FUNCTION "fb_515C_SendData" : VOID
TITLE =Collect the MPI Send signals especial TIE BREAKER
//version!date    !author !change_segm!change_description
//-------+--------+-------+-----------+-------------------------------
// 1.0   !31.08.00!Kahle  ! ---       ! 1st vaild version
// 1.1   !14.11.00!Kahle  ! 1         ! Corr. tie breaker
AUTHOR : Kahle
FAMILY : PMA71
NAME : CollData
VERSION : 1.1


VAR_INPUT
  ONE_TIEBRK : BOOL ;
  IN_Mde_autoOP : BOOL ;	//mode =automatic from OP
END_VAR
VAR_OUTPUT
  IN_Mde_auto : BOOL ;	//mode =automatic from IMAC
END_VAR
VAR_TEMP
  local : BOOL ;	//mode =local
  semiOP : BOOL ;	//mode =semi OP
  autoOP : BOOL ;	//mode =auto OP
  semi : BOOL ;	//mode =semi
  auto : BOOL ;	//mode =auto
  var5 : BOOL ;
  var6 : BOOL ;
  var7 : BOOL ;
END_VAR
BEGIN
NETWORK
TITLE =Collect the MPI Send signals
// c_genBrkOpn, c_unitLock                            ->FB56 "GenProtect"
//
//
// Automatic mode
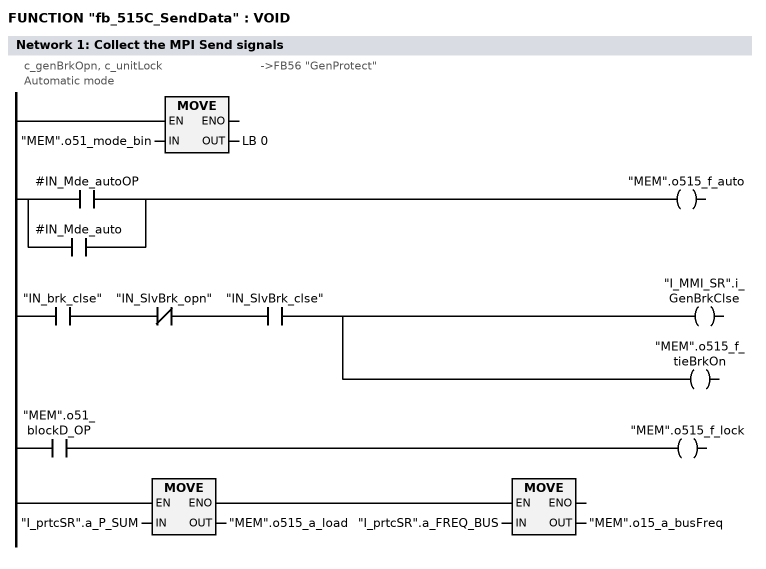
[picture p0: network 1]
      L     "MEM".o51_mode_bin;
      T     LB     0;
      O     #IN_Mde_autoOP;
      O     #IN_Mde_auto;
      =     "MEM".o515_f_auto;

// tie breaker_A close
      U     "IN_brk_clse";
      UN    "IN_SlvBrk_opn";
      U     "IN_SlvBrk_clse";
      =     "I_MMI_SR".i_GenBrkClse;
      =     "MEM".o515_f_tieBrkOn;

// tie breaker A blocked
      O     "MEM".o51_blockD_OP;
      =     "MEM".o515_f_lock;

// actual active load signal
      L     "I_prtcSR".a_P_SUM;
      T     "MEM".o515_a_load;

// actual busbar frequency
      L     "I_prtcSR".a_FREQ_BUS;
      T     "MEM".o15_a_busFreq;

NETWORK
TITLE =no used signal's

      CLR   ;
      =     "MEM".o515_f_brk_clse;

END_FUNCTION



FUNCTION "fc_520_RestoreTie" : VOID
TITLE =Restore tie breaker state after blackout -- ONE tie breaker --
//#### ZERO CALL ####
AUTHOR : Kahle
FAMILY : PMA71
NAME : Rstr1TB
VERSION : 1.0


VAR_INPUT
  FDB_close_A : BOOL ;	//Feedback tie breaker A close
  FDB_open_A : BOOL ;	//Feedback tie breaker A open
  FDB_close_B : BOOL ;	//Feedback tie breaker B close
  FDB_open_B : BOOL ;	//Feedback tie breaker B open
  Blackout_MSB_A : BOOL ;	//backout on main switchboard A
  Blackout_MSB_B : BOOL ;	//blackout on main switchboard B
END_VAR
BEGIN
NETWORK
TITLE =

END_FUNCTION

FUNCTION "fc_TieBrk_shrState" : VOID
TITLE =Determine shore connection state for busbar and transferline
//version!date    !author !change_segm!change_description
//-------+--------+-------+-----------+-------------------------------
// 1.0   !17.07.00!Kahle  ! ---       ! 1st valid version
// 1.1   !13.10.00!Kahle  ! 1(new)    ! Init.int.var.
//       !        !       ! 2         ! Determine the state of foreign tieBrk,
//       !        !       !           ! incl.the other tieBrk of the own station
AUTHOR : Kahle
FAMILY : PMA71
NAME : ShrState
VERSION : 1.1


VAR_INPUT
  IN_synchrToOwnBus : BOOL ;	//Direction of the synchronisation =1: to own bus
  IN_1stTieBrk : BOOL ;	//first tie breaker (=1), sencond tie breaker (=0)
  IN_state_othTieBrk : BOOL ;	//state of the other tie breaker
END_VAR
VAR_OUTPUT
  OUT_shoreBus_on : BOOL ;	//shore connection active at the configuration 1
  OUT_shoreTrs_on : BOOL ;	//shore connection active at the configuration 2
  OUT_SC_Bus : BOOL ;	//short circuit on busbar
  OUT_CfgBusbar : INT ;	//Actual configuration busbar
  OUT_CfgTrans : INT ;	//Actual configuration transferline
END_VAR
VAR_TEMP
  res_0_0 : BOOL ;
  temp_othBrk_TieBrk_1 : BOOL ;	//other breaker of tie breaker controller 1
  temp_othBrk_TieBrk_2 : BOOL ;	//other breaker of tie breaker controller 2
  temp_othBrk_TieBrk_3 : BOOL ;	//other breaker of tie breaker controller 3
  temp_othBrk_TieBrk_4 : BOOL ;	//other breaker of tie breaker controller 4
  res_0_5 : BOOL ;
  res_0_6 : BOOL ;
  res_0_7 : BOOL ;
  temp_tieBrk_1 : BOOL ;	//state of tie breaker 1
  temp_tieBrk_2 : BOOL ;	//state of tie breaker 2
  temp_tieBrk_3 : BOOL ;	//state of tie breaker 3
  temp_tieBrk_4 : BOOL ;	//state of tie breaker 4
  temp_cfg1 : BYTE ;	//actual configuration busbar
  temp_cfg2 : BYTE ;	//actual configuration transferline
  temp_actCfgNo : BYTE ;	//Number of the actual configuration
  temp_actCfgNo_rel : BYTE ;	//Relative number of the actual number
  temp_act_partBus : BYTE ;	//actual bus configuration
  temp_actTieCfg : BYTE ;	//actual tie breaker configuration
  temp_actCfg : DWORD ;	//actual configuration
  temp_rec9 : BYTE ;	//received byte 9 of the actual configration from MPI
END_VAR
BEGIN
NETWORK
TITLE =initalizion of internal variables

      CLR   ;
      =     #temp_othBrk_TieBrk_1;
      =     #temp_othBrk_TieBrk_2;
      =     #temp_othBrk_TieBrk_3;
      =     #temp_othBrk_TieBrk_4;
NETWORK
TITLE =Determine the neighbouring busbar

      L     "prm_pma".p_station;
      +     -1;
      SPL   tie4;
      SPA   tie1;
      SPA   tie2;
      SPA   tie3;
//actual tie breaker =4
tie4: L     4; //part_bus: busbar 4
      L     3; //part_trs: busbar 3
      SPA   cfg;
//actual tie breaker =1
tie1: L     1; //part_bus: busbar 1
      L     2; //part_trs: busbar 2
      SPA   cfg;
//actual tie breaker =2
tie2: L     2; //part_bus: busbar 2
      L     4; //part_trs: busbar 4
      SPA   cfg;
//actual tie breaker =3
tie3: L     3; //part_bus: busbar 1
      L     1; //part_trs: busbar 3
      SPA   cfg;

cfg:  UN    #IN_synchrToOwnBus;
      SPB   stor;
      TAK   ; //if syhchrToOwnBus true then change cfg1 with cfg2
stor: T     #temp_cfg2;
      TAK   ;
      T     #temp_cfg1;

//Check, if the other breaker of the own controller is available
      L     "prm_pma".p_station;
      LAR1  ; //store as pointer "1st breaker"
      UN    #IN_1stTieBrk;
      SPB   chkT;
      +     1;
      LAR1  ; //store as pointer "2nd breaker"
      +     4; //2nd breaker of own station =station address +4 => +1 in int.register
chkT: L     "prm_pma".p_tiebrkCfg;
      SRW   ;
      SPZ   n2nd;

//second tie breaker available
      SET   ;
      =     L [AR1,P#0.0]; //temp_othBrk_TieBrk_'x'

//Determine the state of the foreign tie breakers including the other breaker of the own controller
n2nd: O     "I_tie1SR".f_tieBrkOnT1;
      O(    ;
      U     #IN_state_othTieBrk;
      U     #temp_othBrk_TieBrk_1;
      )     ;
      =     #temp_tieBrk_1;

      O     "I_tie2SR".f_tieBrkOnT2;
      O(    ;
      U     #IN_state_othTieBrk;
      U     #temp_othBrk_TieBrk_2;
      )     ;
      =     #temp_tieBrk_2;

      O     "I_tie3SR".f_tieBrkOnT3;
      O(    ;
      U     #IN_state_othTieBrk;
      U     #temp_othBrk_TieBrk_3;
      )     ;
      =     #temp_tieBrk_3;

      O     "I_tie4SR".f_tieBrkOnT4;
      O(    ;
      U     #IN_state_othTieBrk;
      U     #temp_othBrk_TieBrk_4;
      )     ;
      =     #temp_tieBrk_4;

//*********************************************************************************************************
//****   BUSBAR                                                                                        ****
//*********************************************************************************************************

//Determine the actual configuration 'busbar'
      CALL "fc_93_CnfgDecod" (
           tieBrk_1                 := #temp_tieBrk_1,
           tieBrk_2                 := #temp_tieBrk_2,
           tieBrk_3                 := #temp_tieBrk_3,
           tieBrk_4                 := #temp_tieBrk_4,
           tieBrkHW_1               := "IN_tieBrk_1",
           tieBrkHW_2               := "IN_tieBrk_2",
           tieBrkHW_3               := "IN_tieBrk_3",
           tieBrkHW_4               := "IN_tieBrk_4",
           partBusNo                := #temp_cfg1,
           actCfgNo                 := #temp_actCfgNo,
           actCfgNo_rel             := #temp_actCfgNo_rel,
           act_partBus              := #temp_act_partBus,
           actTieCfg                := #temp_actTieCfg);

      L     #temp_actCfgNo_rel;
      SLW   4; //convert to pointer *2 (=INT)
      LAR1  ;
      AUF   "prm_pma";
      L     DBW [AR1,P#6.0];
      T     #OUT_CfgBusbar; //Actual configuration busbar
      L     W#16#C000;
      UW    ; //shore connection only
      SLD   4;
      T     #temp_actCfg; //actual bus configuration

//Check if on the busbar side a shore connection on
//Received commands from Gen 1 -13, EG, TieBrk 1-4, Shore1,2 (D39.2, D39.5 -D 39.7) <OR>
      CALL "fc_95_fdbHndl" (
           IN_off                   := B#16#9,
           IN_mask                  := B#16#0,// bit0 -7: OR
           IN_release               := #temp_actCfg,
           OUT_fdb                  := #temp_rec9);//received MPI commands (byte 9)
      L     #temp_rec9;
      CLR   ;
      SRW   6;
      SPZ   shr1;
      SET   ;
shr1: =     #OUT_shoreBus_on;

      L     #OUT_CfgBusbar; //Actual configuration busbar
      SLD   4;
      T     #temp_actCfg; //actual bus configuration

//Check if on the busbar side a shore connection on
//Received commands from Gen 1 -13, EG, TieBrk 1-4, Shore1,2 (D39.2, D39.5 -D 39.7) <OR>
      CALL "fc_95_fdbHndl" (
           IN_off                   := B#16#9,
           IN_mask                  := B#16#0,// bit0 -7: OR
           IN_release               := #temp_actCfg,
           OUT_fdb                  := #temp_rec9);//received MPI commands (byte 9)
      L     #temp_rec9;
      CLR   ;
      SRW   3;
      SPZ   shrt;
      SET   ;
shrt: =     #OUT_SC_Bus;

//*********************************************************************************************************
//****   TRANSFERLINE                                                                                  ****
//*********************************************************************************************************

//Determine the actual configuration 'transferline'
      CALL "fc_93_CnfgDecod" (
           tieBrk_1                 := #temp_tieBrk_1,
           tieBrk_2                 := #temp_tieBrk_2,
           tieBrk_3                 := #temp_tieBrk_3,
           tieBrk_4                 := #temp_tieBrk_4,
           tieBrkHW_1               := "IN_tieBrk_1",
           tieBrkHW_2               := "IN_tieBrk_2",
           tieBrkHW_3               := "IN_tieBrk_3",//convert to pointer *2 (=INT)
           tieBrkHW_4               := "IN_tieBrk_4",
           partBusNo                := #temp_cfg2,
           actCfgNo                 := #temp_actCfgNo,
           actCfgNo_rel             := #temp_actCfgNo_rel,
           act_partBus              := #temp_act_partBus,//shore connection only
           actTieCfg                := #temp_actTieCfg);

      L     #temp_actCfgNo_rel; //actual bus configuration
      SLW   4; //Actual configuration transferline
      LAR1  ;
      AUF   "prm_pma";
      L     DBW [AR1,P#6.0]; // bit0 -7: OR
      T     #OUT_CfgTrans;
      L     W#16#C000;
      UW    ; //received MPI commands (byte 9)
      SLD   4;
      T     #temp_actCfg;

//Check if on the transferline side a shore connection on
//Received commands from Shore1,2 (39.7) <OR>
      CALL "fc_95_fdbHndl" (
           IN_off                   := B#16#9,
           IN_mask                  := B#16#0,// bit0 -7: OR
           IN_release               := #temp_actCfg,
           OUT_fdb                  := #temp_rec9);//received MPI commands (byte 9)
      L     #temp_rec9;
      CLR   ;
      SRW   6;
      SPZ   shr2;
      SET   ;
shr2: =     #OUT_shoreTrs_on;
END_FUNCTION



FUNCTION "fc_TieBrk_StandbyStrt" : VOID
TITLE =Standby Start in case of overcurrent tie breaker
AUTHOR : Kahle
FAMILY : PMA71
NAME : StdStrtT
VERSION : 1.0


VAR_INPUT
  IN_load : INT ;	//Actual load [in kW]
  IN_CfgBusbar : INT ;	//Actual configuration busbar
  IN_CfgTrans : INT ;	//Actual configuration transferline
END_VAR
VAR_OUTPUT
  temp_stdbyNo : BYTE ;	//Nummer of the actual standby generator set
END_VAR
VAR_TEMP
  temp_actCfg : WORD ;	//Actual configuration
  x : BYTE ;
  xx : BOOL ;
  temp_code1_8 : DINT ;
  temp_code9_15 : DINT ;
END_VAR
BEGIN
NETWORK
TITLE =Determine the conduction direction

      L     #IN_load;
      L     0;
      <I    ;
      L     #IN_CfgBusbar; //p <0 ...standby start busbar
      SPB   busB;
      L     #IN_CfgTrans; //p >0 ...standby start transferline
busB: T     #temp_actCfg;
NETWORK
TITLE =Determine the actual start/stop sequence

      CALL "fc_92_SelctCnfg" (
           start                    := TRUE,
           code_gen_1               := "MEM".o51_code1_8,
           code_gen_2               := "MEM".o51_code9_15,
           act_cfg                  := #temp_actCfg,
           code_gen1_act            := #temp_code1_8,
           code_gen2_act            := #temp_code9_15);

NETWORK
TITLE =Detemine the standby diesel (actual configuration)

      CALL "fc_52_preselect" (
           IN_gen1_8                := #temp_code1_8,
           IN_gen9_15               := #temp_code9_15,
           IN_ownStat               := B#16#0,
           IN_binMode               := B#16#0,
           IN_ready                 := FALSE,
           IN_running               := FALSE,
           IN_StpForbid             := FALSE,
           OUT_stdby_1st            := #xx,
           OUT_stdby_2nd            := #xx,
           OUT_stdbyNo_1st          := #temp_stdbyNo,
           OUT_stdbyNo_2nd          := #x,
           OUT_SD                   := #xx,
           OUT_SDNo                 := #x);


END_FUNCTION


FUNCTION "fc_h24_ABS(INT)" : VOID
TITLE =absolute value
AUTHOR : Kahle
FAMILY : PMA71
NAME : ABS_INT
VERSION : 1.0


VAR_INPUT
  IN_value : INT ;
END_VAR
VAR_OUTPUT
  OUT_absValue : INT ;
END_VAR
VAR_TEMP
  temp_val_x8 : BOOL ;
  temp_val_x9 : BOOL ;
  temp_val_x10 : BOOL ;
  temp_val_x11 : BOOL ;
  temp_val_x12 : BOOL ;
  temp_val_x13 : BOOL ;
  temp_val_x14 : BOOL ;
  temp_val_x15 : BOOL ;
  temp_val_x0 : BOOL ;
  temp_val_x1 : BOOL ;
  temp_val_x2 : BOOL ;
  temp_val_x3 : BOOL ;
  temp_val_x4 : BOOL ;
  temp_val_x5 : BOOL ;
  temp_val_x6 : BOOL ;
  temp_val_x7 : BOOL ;
END_VAR
BEGIN
NETWORK
TITLE =

      L     #IN_value;
      T     LW     0;

      U     #temp_val_x15; //if value not negative ...jump
      SPBN  out;
      NEGI  ;
out:  T     #OUT_absValue;
END_FUNCTION


FUNCTION "fc_h20_NoParticip" : VOID
TITLE =Number of a signal of all participants
//
//                                                                             !
//The function list a signal over all defined participants
AUTHOR : Kahle
FAMILY : PMA71
NAME : fdbHandl
VERSION : 1.1


VAR_INPUT
  IN_bytebit : POINTER ;	//relative byte.bit address
  IN_release : WORD ;	//release source (bit0 =1:release 1.gen., ..bit12 =1:release 13.gen.
END_VAR
VAR_OUTPUT
  OUT_Signal_No : INT ;	//Number of signals
  OUT_GenSetOnbus : WORD ;
END_VAR
VAR_TEMP
  source : INT ;	//last source address
  cnt_coll : BYTE ;	//loop counter 'collected signals'
  Signal_No : BYTE ;	//temporary memory numbers of signal over all participants
  genSet_onbus : WORD ;	//generator sets on busbar (breaker close)
END_VAR
BEGIN
NETWORK
TITLE =intial. internal signals
//
//
      L     0;
      T     #genSet_onbus;
      L     122;
      T     #source; //last generator DB
      L     30;
      L     P##IN_bytebit;
      LAR1  ;
      L     D [AR1,P#2.0];
      LAR1  ; //source byte address
      L     0;
      T     #Signal_No;

NETWORK
TITLE =collect the signals from the generators

      L     14; //start =last source
lpco: T     #cnt_coll;
      L     #IN_release;
      SRW   ;
      SPZ   nxco; //if release gen(#cnt_coll) =false then ..next generator

//source =own station
      L     "prm_pma".p_station;
      +     -4;
      L     #cnt_coll;
      ==I   ;
      SPB   nxco; //if source station =own station then ...next generator

//list the signal over all participants
      AUF   DB [#source];
      UN    DBX [AR1,P#0.0];
      SPB   nxco; //signal (byte.bit) false ...next participant

      L     #Signal_No;
      +     1;
      T     #Signal_No; //add up

//generator sets on busbar
      L     #cnt_coll;
      L     DW#16#80000000;
      RLD   ;
      L     #genSet_onbus;
      OW    ;
      T     #genSet_onbus;

//next generator
nxco: L     #source;
      +     -1;
      T     #source; //next step ->next source
      L     #cnt_coll;
      LOOP  lpco;

//output
      L     #Signal_No;
      T     #OUT_Signal_No;
      L     #genSet_onbus;
      T     #OUT_GenSetOnbus;
END_FUNCTION


FUNCTION_BLOCK "StartGenSet"
TITLE =Start a defined Generatorset
AUTHOR : Kahle
FAMILY : PMA71
NAME : StrtGenS
VERSION : 1.0


VAR_INPUT
  IN_start : BOOL ;	//Start command
  IN_destGen : BYTE ;	//destination generator set
  IN_time : S5TIME ;	//time of start signal is activing
  IN_timerNo : TIMER ;	//Timer number
END_VAR
VAR_OUTPUT
  OUT_sendPulse : BOOL ;
END_VAR
VAR
  stat_step : BYTE ;
  stat_destGen : BYTE ;
  stat_startPulse : BOOL ;
  stat_sendSignal : BOOL ;
  stat_pulseStep1 : BOOL ;
  stat_pulseStep2 : BOOL ;
END_VAR
VAR_TEMP
  temp_destDB : WORD ;
END_VAR
BEGIN
NETWORK
TITLE =Step_1 preconditions

      U(    ;
      U     #IN_start;
      FP    #stat_startPulse;
      )     ;
      U(    ;
      L     #stat_step;
      L     0;
      ==I   ;
      )     ;
      SPBN  sp1c;
      L     1;
      T     #stat_step;
NETWORK
TITLE =Step_1 commands

sp1c: L     #stat_step;
      L     1;
      ==I   ;
      =     #stat_sendSignal;
      FP    #stat_pulseStep1;
      SPBN  sp2p;
      L     #IN_time;
      CLR   ;
      SV    #IN_timerNo;
      SET   ;
      SV    #IN_timerNo;
      L     #IN_destGen;
      T     #stat_destGen;
NETWORK
TITLE =step_2 preconditions

sp2p: UN    #IN_timerNo;
      U(    ;
      L     #stat_step;
      L     1;
      ==I   ;
      )     ;
      SPBN  sp2c;
      L     2;
      T     #stat_step;

NETWORK
TITLE =step_2 commands

sp2c: L     #stat_step;
      L     2;
      ==I   ;
      FP    #stat_pulseStep2;
      SPBN  st3p;
      L     #IN_time;
      CLR   ;
      SV    #IN_timerNo;
      SET   ;
      SV    #IN_timerNo;


NETWORK
TITLE =step_3 preconditions
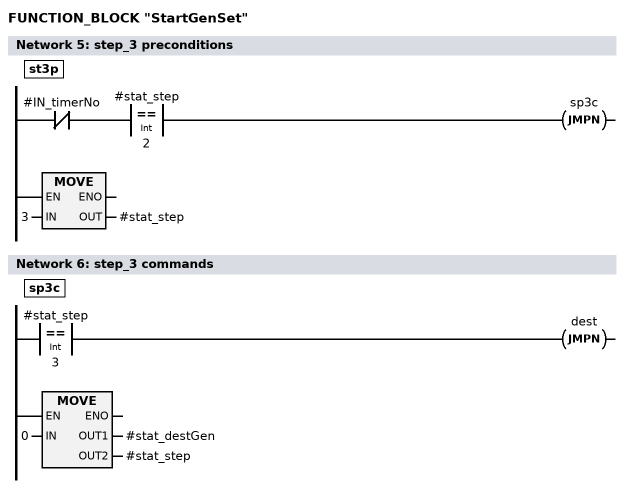
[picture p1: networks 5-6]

st3p: UN    #IN_timerNo;
      U(    ;
      L     #stat_step;
      L     2;
      ==I   ;
      )     ;
      SPBN  sp3c;
      L     3;
      T     #stat_step;


NETWORK
TITLE =step_3 commands

sp3c: L     #stat_step;
      L     3;
      ==I   ;
      SPBN  dest;
      L     0;
      T     #stat_destGen;
      T     #stat_step;
NETWORK
TITLE =send start pulse to the actual generator set

dest: U     #stat_sendSignal;
      =     #OUT_sendPulse;

      L     0;
      L     #stat_destGen;
      ==I   ;
      BEB   ; //no destination ->end
      +     108; //offset Send_DB 'actual destination'
      T     #temp_destDB;
      AUF   DB [#temp_destDB];
      U     #stat_sendSignal;
      =     DBX    0.5; //remote start generator set
END_FUNCTION_BLOCK

FUNCTION_BLOCK "fb_520_tieBreaker"
TITLE =Tie breaker monitoring
//This program controlled the following functions:
//
// - Check the release conditions
// - Lock / release the controller in the generator sets
// - Monitoring of the shutdown criteria
//
//version!date    !author !change_segm!change_description
//-------+--------+-------+-----------+-------------------------------
// 1.0   !26.03.00!Kahle  ! ---       ! 1st version
// 1.1   !28.04.00!Kahle  ! 34        ! Release criteria: shore conn.on
//       !        !       ! 35(new)   ! Alarm "shore conn.on"
//       !        !       ! 19        ! Store rest delay time
//       !        !       ! 39(new)   ! Recover breaker state after blackout
//       !        !       ! 40        ! Parameter "IN_PB_GenBrk_close": add.signal
// 1.2   !17.05.00!Kahle  ! 34,36     ! Blocked in case of shore connection if
//       !        !       !           ! no blackout transferline only
//       !        !       ! 19,20,40  ! Blackout dedecting time
// 1.3   !13.07.00!Kahle  ! 40,41     ! Restore tie breaker delete
//       !        !       ! 19        ! blackout MSB indication
// 1.4   !24.07.00!Kahle  ! 23        ! Indication "blackout both sides"
// 1.5   !31.07.00!Kahle  ! 36,38     ! Both shore =export then no blocked
// 1.6   !25.09.00!Kahle  ! 19,21     ! Corr.Parameter p_Vblackout,p_Tblackout,
//       !        !       !           ! p_TFBusbar
// 1.7   !13.10.00!Kahle  ! IN        ! new parameter 'IN_othBrk_on'
//       !        !       ! 4         ! new parameter 'IN_1stTieBrk'
//       !        !       !           !               'IN_state_othTieBrk'
// 1.8   !14.11.00!Kahle  ! 38        ! as cfg =11 no external release
//       !        !       ! 41        ! slave breaker off, then open tie breaker
// 1.9   !08.12.00!Kahle  ! 38        ! corr. cfg =11: no external release
// 1.10  !10.01.01!Kahle  ! 23        ! corr. ind'blackout busbar'
//       !        !       ! 5         ! ind.'cfg.busbar'
// 1.11  !14.03.01!Kahle  ! 22        ! in_FB_GenBrk_On if no blocking active
//       !        !       !           ! new alarm: overcurrent, overload
//       !        !       ! 41        ! in_DI_GenBrk_NormPos if no blocking active
//       !        !       !           ! in_DI_GenBrk_TestPos if no blocking active
//       !        !       !           ! in_ext_DG_block new
AUTHOR : Kahle
FAMILY : PMA71
NAME : TieMonit
VERSION : 1.11


VAR_INPUT
  IN_synchrToOwnBus : BOOL ;	//Direction of the synchronisation =1: to own bus
  IN_cmd_TieBrk_on : BOOL ;	//Command tie breaker on
  IN_cmd_TieBrk_off : BOOL ;	//Command tie breaker off
  IN_PB_TieBrk_off : BOOL ;	//PB tie breaker off
  IN_blackout_bus : BOOL ;	//Blackout detected on the busbar
  IN_VoltAvail_bus : BOOL ;	//Voltage available on the busbar
  IN_blackout_TRS : BOOL ;	//Blackout detected on the transferline
  IN_VoltAvail_TRS : BOOL ;	//Voltage available on the transferline
  IN_slaveBrk_on : BOOL ;	//slave tie breaker is closed
  IN_shoreConnBus_active : BOOL ;	//shore connection busbar is active
  IN_shoreConnTrs_active : BOOL ;	//shore connection transferline is active
  IN_both_shore_exp : BOOL ;	//both shore connection direction =export
  IN_shortCircuit_otherG : BOOL ;	//At least one generator set has a short circuit detected
  IN_shortCircuit_ext : BOOL ;	//External device has a short circuit dedected
  IN_GEN_I_L1 : INT ;	//GENOP71: I_L1
  IN_GEN_I_L2 : INT ;	//GENOP71: I_L2
  IN_GEN_I_L3 : INT ;	//GENOP71: I_L3
  IN_LOAD : INT ;	//GENOP71: active power [in kW]
  IN_BUS_f : INT ;	//GENOP71: f_bus
  IN_GEN_f : INT ;	//GENOP71: f_gen
  IN_BUS_U_L1L2 : INT ;	//GENOP71: U_L1L2_bus
  IN_BUS_U_L2L3 : INT ;	//GENOP71: U_L2L3_bus
  IN_BUS_U_L1L3 : INT ;	//GENOP71: U_L1L3_bus
  IN_GEN_U_L1L21 : INT ;	//GENOP71: U_L1L2_gen
  IN_GEN_U_L2L31 : INT ;	//GENOP71: U_L2L3_gen
  IN_GEN_U_L1L31 : INT ;	//GENOP71: U_L1L3_gen
  IN_I_SC_GW1 : BOOL ;	//GENOP71: I_SC_GW1
  IN_I_GW1VER : BOOL ;	//GENOP71: I_GW1VER
  IN_I_GW2VER : BOOL ;	//GENOP71: I_GW2VER
  IN_I_GW3VER : BOOL ;	//GENOP71: I_GW3VER
  IN_I_GW4VER : BOOL ;	//GENOP71: I_GW4VER
  IN_simLock_blc : BOOL ;	//Simultaneous lock is blocked
  IN_simLock_err : BOOL ;	//Simultaneous lock failure
  IN_simLockRel : BOOL ;	//Simultaneous lock release
  IN_brk_ready : BOOL ;	//Breaker is ready for closing
  IN_brk_normPos : BOOL ;	//Breaker is in norm position
  IN_brk_testPos : BOOL ;	//Breaker is in test position
  IN_brk_on : BOOL ;	//Feedback: breaker is on
  IN_brk_off : BOOL ;	//Feedback: breaker is off
  IN_othBrk_on : BOOL ;	//Feedback: other breaker is on (second one)
  IN_f_cmdBrkOn : BOOL ;	//Genop Feedback: command breaker on
  IN_reset : BOOL ;	//Reset command
  IN_resetBlock : BOOL ;	//Reset blocking
  IN_pressCnfrm : BOOL ;	//indication: press confirmation
  IN_mode : BYTE ;	//Actual mode (x.0:local, x.1:semiOP, x.2:autoOP, x.3:semi, x.4:auto, x.5:test)
  IN_TimerStdbyStrt : TIMER ;	//Timer startpulse "standby start"
  IN_TimerOpnBrk4Gen : TIMER ;	//Timer delay time befor opening tie breaker in case of 4 running generator sets
END_VAR
VAR_OUTPUT
  OUT_SynchrActive : BOOL ;	//Command: switch up/down
  OUT_c_LckCtrl : BOOL ;	//Command: controller lock
  OUT_c_simLock : BOOL ;	//Command: simultanoeus lock active
  OUT_c_brkON : BOOL ;	//GENOP Command: breaker on
  OUT_c_brkOFF : BOOL ;	//GENOP Command: breaker off
  OUT_c_synRel : BOOL ;	//GENOP Command: synchronizing release
  OUT_c_reqStrt : BOOL ;	//Command: request standby start
  OUT_c_sc_otherSet : BOOL ;	//Command "block set; open tie breaker" in case of a short circuit
  OUT_i_blocked : BOOL ;	//Indication: tie breaker is blocked
  OUT_i_blackout_busbar : BOOL ;	//Indication: blackout busbar
  OUT_i_blackout_trans : BOOL ;	//Indication: blackout transferline
  OUT_i_CfgBusbar : INT ;	//Indication: actual configuration busbar
  OUT_e_transfer_monit : BOOL ;	//Failure: transfer line monitoring
  OUT_e_busbar_monit : BOOL ;	//Failure: busbar monitoring
  OUT_e_I_monit : BOOL ;	//Failure: current monitoring
  OUT_e_I_trip : BOOL ;	//Failure: tripped by overcurrent
  OUT_e_I : BOOL ;	//Warning: overcurrent
  OUT_e_P : BOOL ;	//Warning: overload
  OUT_e_f1 : BOOL ;	//Failure: underfrequency 1
  OUT_e_f2 : BOOL ;	//Failure: underfrequency 2
  OUT_e_f3 : BOOL ;	//Failure: underfrequency 3
  OUT_e_f4 : BOOL ;	//Failure: overfrequency
  OUT_e_U1 : BOOL ;	//Failure: undervoltage 1
  OUT_e_U2 : BOOL ;	//Failure: undervoltage 2
  OUT_e_U3 : BOOL ;	//Failure: undervoltage 3
  OUT_e_U4 : BOOL ;	//Failure: overvoltage
  OUT_e_I_sc : BOOL ;	//Failure: short circuit
  OUT_e_sc_other : BOOL ;	//Failure: short circuit at other generator set
  OUT_e_black : BOOL ;	//Failure: blackout
  OUT_e_brkRdy : BOOL ;	//Failure: breaker ready
  OUT_e_brkOn : BOOL ;	//Failure: breaker on
  OUT_e_brkOff : BOOL ;	//Failure: breaker off
  OUT_e_brkOnOff : BOOL ;	//Failure: breaker feedbak plausibility
  OUT_e_brkTrip : BOOL ;	//Failure: breaker tripped
  OUT_e_synTime : BOOL ;	//Failure: synchronization time exceeded
  OUT_e_StdbyStart : BOOL ;	//Failure: standby start
  OUT_e_ShoreActive : BOOL ;	//Failure: shore connection is active, synchronizing not possible
  OUT_ind_ready : BYTE ;	//indication: criteria for breaker ready
  OUT_ind_line1_stat : INT ;	//status indication -line 1-
  out_ind_line2_var : INT ;	//status indication -line 2-
END_VAR
VAR
  Gen_Protect : "fb_511_GenProtect";
  Gen_Breaker : "fb_57_clseopnBrk";
  RemoteStart : "StartGenSet";
  BlockTieBrk : BOOL ;	//Tie breaker is blocked
  BothSideBlackout : BOOL ;	//Blackout on the entire busbar
  tieBrk_state : BOOL ;	//State of the tie breaker (=0:open, =1:close)
  pulse_SlvBrk : BOOL ;	//Flag "slave braker state"
  Generator_Protect : "fb_511_GenProtect";	//Generator protection
  Breaker_control : "fb_57_clseopnBrk";	//Breaker control (close, open, monitoring)
  memo_GenSetOnBus : WORD ;
  memo_newGenSet : WORD ;
END_VAR
VAR_TEMP
  temp_OM_Local : BOOL ;	//Active operation mode: Local
  temp_OM_Semi_OP : BOOL ;	//Active operation mode: Semi automatic OP
  temp_OM_Auto_OP : BOOL ;	//Active operation mode: Automatic OP
  temp_OM_Semi_MMI : BOOL ;	//Active operation mode: Semi automatic MMI
  temp_OM_Auto_MMI : BOOL ;	//Active operation mode: Automatic MMI
  temp_OM_Test : BOOL ;	//Active operation mode: Test (EG only)
  temp_Reserve_006 : BOOL ;	//Reserved (Transfer Byte --> Bit)
  temp_Reserve_007 : BOOL ;	//Reserved (Transfer Byte --> Bit)
  temp_OM_Local_Prt : BOOL ;	//Active operation mode: Local
  temp_OM_Semi_OP_Prt : BOOL ;	//Active operation mode: Semi automatic OP
  temp_OM_Auto_OP_Prt : BOOL ;	//Active operation mode: Automatic OP
  temp_OM_Semi_MMI_Prt : BOOL ;	//Active operation mode: Semi automatic MMI
  temp_OM_Auto_MMI_Prt : BOOL ;	//Active operation mode: Automatic MMI
  temp_OM_Test_Prt : BOOL ;	//Active operation mode: Test (EG only)
  temp_Reserve_006_Prt : BOOL ;	//Reserved (Transfer Byte --> Bit)
  temp_Reserve_007_Prt : BOOL ;	//Reserved (Transfer Byte --> Bit)
  temp_ext_release : BOOL ;	//external releases
  temp_shoreTrs_on : BOOL ;	//shore connection active at the configuration 2
  temp_blackBus : BOOL ;	//blackout on the busbar
  temp_blackTrans : BOOL ;	//blackout on the transferline
  temp_blackout : BOOL ;	//blackout on busbar/ transferline
  temp_TieOffBlack : BOOL ;	//On side blackout: tie breaker off
  temp_TieOffNoGen : BOOL ;	//Number of allowed generator exceeded: tie breaker off
  temp_req_StdbyStrt : BOOL ;	//Request start standby generator set
  temp_Brk_off : BOOL ;	//Command: breaker off
  temp_block : BOOL ;	//Blocking own breaker
  temp_Auto : BOOL ;	//mode =automatic OP or automatic MMI
  temp_tieBrk_ready : BOOL ;	//tie breaker ready
  var24 : BOOL ;
  var25 : BOOL ;
  var26 : BOOL ;
  var27 : BOOL ;
  temp_slaveBrk_on : BOOL ;	//slave breaker on
  temp_blackBlock : BOOL ;	//blackout on both busbar
  temp_VoltAvailBus : BOOL ;	//Busbar voltage available
  temp_shoreBus_on : BOOL ;	//shore connection active at the configuration 1
  temp_shoreTrs_off : BOOL ;	//shore connection not active at the configuration 2
  temp_Semi : BOOL ;	//Active operation mode: Semi automatic
  temp_normTestPos : BOOL ;	//Breaker in norm or test position
  temp_readyClose : BOOL ;	//Breaker is ready for closing
  temp_voltAvailPrtct : BOOL ;	//Voltage on busbar or transferline available (protetion unit)
  temp_VoltAvailTrs : BOOL ;	//Transferline voltage available
  temp_GEN_I_L1 : INT ;	//Generator current L1 (in 100.00% of nominal value)
  temp_GEN_I_L2 : INT ;	//Generator current L1 (in 100.00% of nominal value)
  temp_GEN_I_L3 : INT ;	//Generator current L1 (in 100.00% of nominal value)
  temp_BUS_f : INT ;	//Bus bar frequency (in 100.00% of nominal value)
  temp_GEN_f : INT ;	//Generator frequency (in 100.00% of nominal value)
  temp_BUS_U_L1L2 : INT ;	//Bus bar voltage L1/L2 (in 100.00% of nominal value)
  temp_BUS_U_L2L3 : INT ;	//Bus bar voltage L2/L3 (in 100.00% of nominal value)
  temp_BUS_U_L3L1 : INT ;	//Bus bar voltage L3/L1 (in 100.00% of nominal value)
  temp_GEN_U_L1L2 : INT ;	//Generator voltage L1/L2 (in 100.00% of nominal value)
  temp_GEN_U_L2L3 : INT ;	//Generator voltage L2/L3 (in 100.00% of nominal value)
  temp_GEN_U_L3L1 : INT ;	//Generator voltage L3/L1 (in 100.00% of nominal value)
  temp_GEN_P_SUM : INT ;	//Generator active load (in 100.00% of nominal value)
  temp_GenNo_onbus : INT ;	//Number of generator which are on busbar
  temp_CfgBusbar : INT ;	//Actual configration busbar
  temp_CfgTrans : INT ;	//Actual configuration transferline
  temp_Indication2_FB51 : INT ;	//Indication number, line 2, from FB51
  temp_Operat_Status : INT ;	//status indication for OP7
  temp_GenSetOnbus : WORD ;
  temp_GenSetOwn : BOOL ;
  temp_SC_busbar : BOOL ;	//short circuit on busbar
  temp_blackout_undly : BOOL ;	//blackout undelayed
  temp_blackoutT_run : BOOL ;	//blackout detecting time is running
  temp_stdbyNo_1st : BYTE ;	//Number of the actual standby generator
  temp_GEN_U_Max : INT ;	//Mains (generator) voltage, highest value (phase L1/L2, L2/L3, L3/L1)
  temp_RdlyTrun_blackBus : WORD ;	//Rest of the delay time "blackout busbar"
END_VAR
BEGIN
NETWORK
TITLE =Active operation mode (Transfer Byte --> Bit)
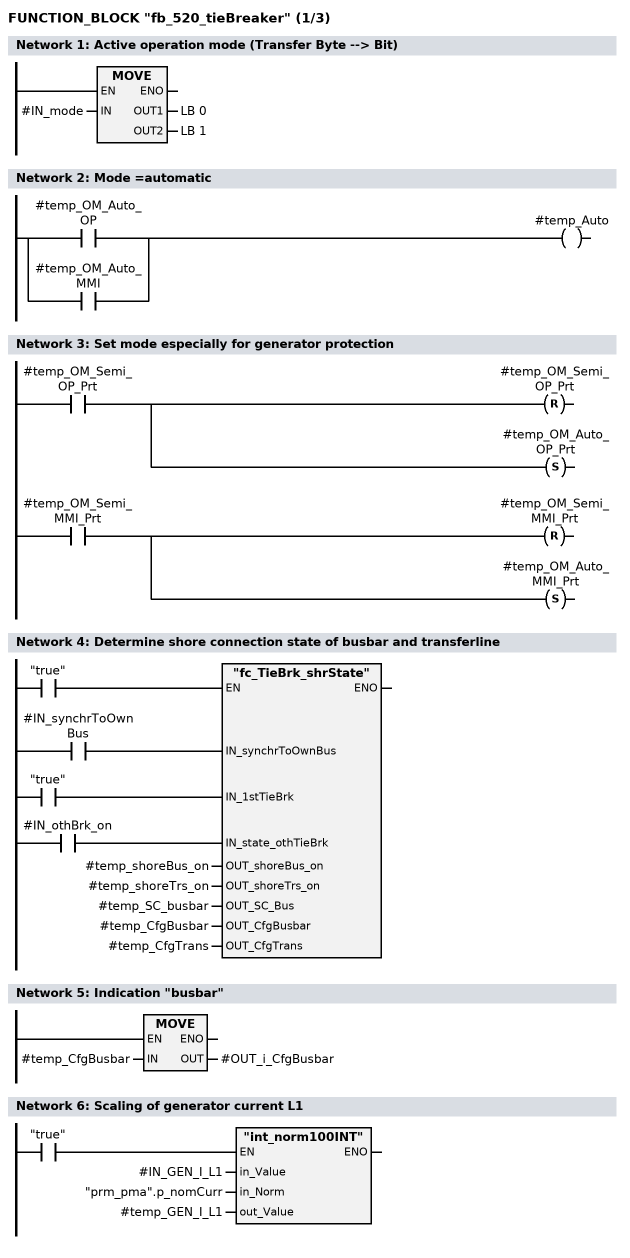
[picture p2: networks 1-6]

      L     #IN_mode;
      T     LB     0;
      T     LB     1;
NETWORK
TITLE =Mode =automatic

      O     #temp_OM_Auto_OP;
      O     #temp_OM_Auto_MMI;
      =     #temp_Auto;
NETWORK
TITLE =Set mode especially for generator protection

      U     #temp_OM_Semi_OP_Prt;
      R     #temp_OM_Semi_OP_Prt;
      S     #temp_OM_Auto_OP_Prt;

      U     #temp_OM_Semi_MMI_Prt;
      R     #temp_OM_Semi_MMI_Prt;
      S     #temp_OM_Auto_MMI_Prt;
NETWORK
TITLE =Determine shore connection state of busbar and transferline

      U     #IN_synchrToOwnBus;
      =     L     48.0;
      BLD   103;
      U     "true";
      =     L     48.1;
      BLD   103;
      U     #IN_othBrk_on;
      =     L     48.2;
      BLD   103;
      U     "true";
      SPBNB _001;
      CALL "fc_TieBrk_shrState" (
           IN_synchrToOwnBus        := L     48.0,
           IN_1stTieBrk             := L     48.1,
           IN_state_othTieBrk       := L     48.2,
           OUT_shoreBus_on          := #temp_shoreBus_on,
           OUT_shoreTrs_on          := #temp_shoreTrs_on,
           OUT_SC_Bus               := #temp_SC_busbar,
           OUT_CfgBusbar            := #temp_CfgBusbar,
           OUT_CfgTrans             := #temp_CfgTrans);
_001: NOP   0;
NETWORK
TITLE =Indication "busbar"

      L     #temp_CfgBusbar;
      T     #OUT_i_CfgBusbar;
NETWORK
TITLE =Scaling of generator current L1

      U     "true";
      SPBNB _002;
      CALL "int_norm100INT" (
           in_Value                 := #IN_GEN_I_L1,
           in_Norm                  := "prm_pma".p_nomCurr,
           out_Value                := #temp_GEN_I_L1);
_002: NOP   0;
NETWORK
TITLE =Scaling of generator current L2
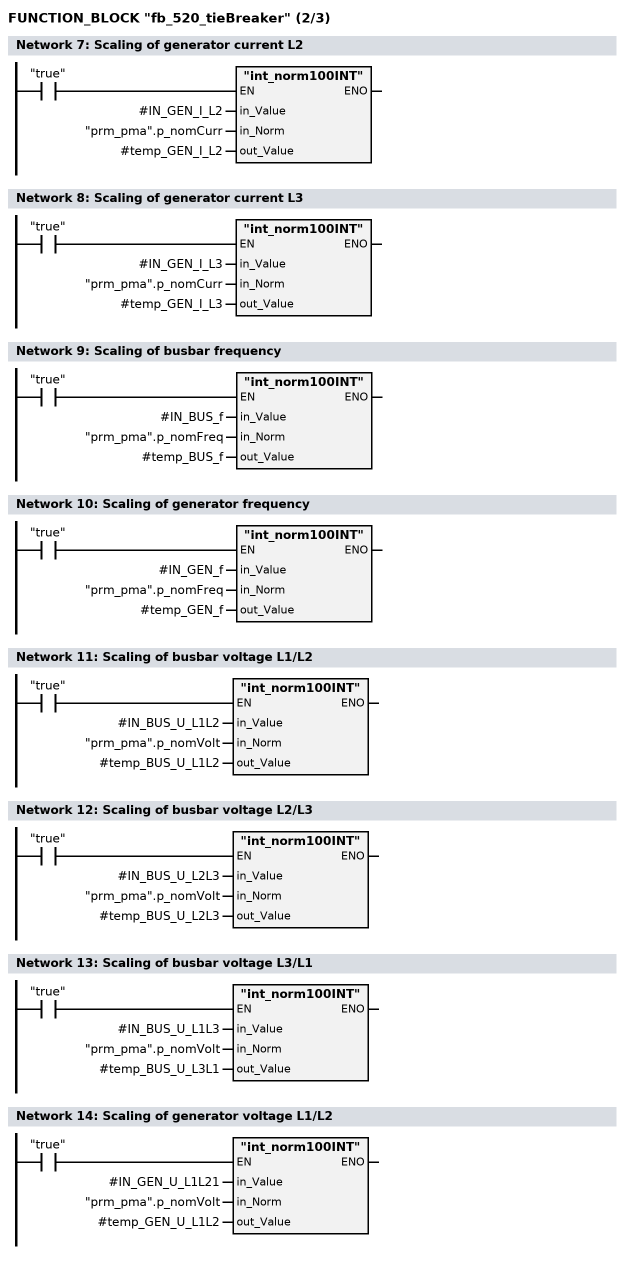
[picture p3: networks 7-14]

      U     "true";
      SPBNB _003;
      CALL "int_norm100INT" (
           in_Value                 := #IN_GEN_I_L2,
           in_Norm                  := "prm_pma".p_nomCurr,
           out_Value                := #temp_GEN_I_L2);
_003: NOP   0;
NETWORK
TITLE =Scaling of generator current L3

      U     "true";
      SPBNB _004;
      CALL "int_norm100INT" (
           in_Value                 := #IN_GEN_I_L3,
           in_Norm                  := "prm_pma".p_nomCurr,
           out_Value                := #temp_GEN_I_L3);
_004: NOP   0;
NETWORK
TITLE =Scaling of busbar frequency

      U     "true";
      SPBNB _005;
      CALL "int_norm100INT" (
           in_Value                 := #IN_BUS_f,
           in_Norm                  := "prm_pma".p_nomFreq,
           out_Value                := #temp_BUS_f);
_005: NOP   0;
NETWORK
TITLE =Scaling of generator frequency

      U     "true";
      SPBNB _006;
      CALL "int_norm100INT" (
           in_Value                 := #IN_GEN_f,
           in_Norm                  := "prm_pma".p_nomFreq,
           out_Value                := #temp_GEN_f);
_006: NOP   0;
NETWORK
TITLE =Scaling of busbar voltage L1/L2

      U     "true";
      SPBNB _007;
      CALL "int_norm100INT" (
           in_Value                 := #IN_BUS_U_L1L2,
           in_Norm                  := "prm_pma".p_nomVolt,
           out_Value                := #temp_BUS_U_L1L2);
_007: NOP   0;
NETWORK
TITLE =Scaling of busbar voltage L2/L3

      U     "true";
      SPBNB _008;
      CALL "int_norm100INT" (
           in_Value                 := #IN_BUS_U_L2L3,
           in_Norm                  := "prm_pma".p_nomVolt,
           out_Value                := #temp_BUS_U_L2L3);
_008: NOP   0;
NETWORK
TITLE =Scaling of busbar voltage L3/L1

      U     "true";
      SPBNB _009;
      CALL "int_norm100INT" (
           in_Value                 := #IN_BUS_U_L1L3,
           in_Norm                  := "prm_pma".p_nomVolt,
           out_Value                := #temp_BUS_U_L3L1);
_009: NOP   0;
NETWORK
TITLE =Scaling of generator voltage L1/L2

      U     "true";
      SPBNB _00a;
      CALL "int_norm100INT" (
           in_Value                 := #IN_GEN_U_L1L21,
           in_Norm                  := "prm_pma".p_nomVolt,
           out_Value                := #temp_GEN_U_L1L2);
_00a: NOP   0;
NETWORK
TITLE =Scaling of generator voltage L2/L3
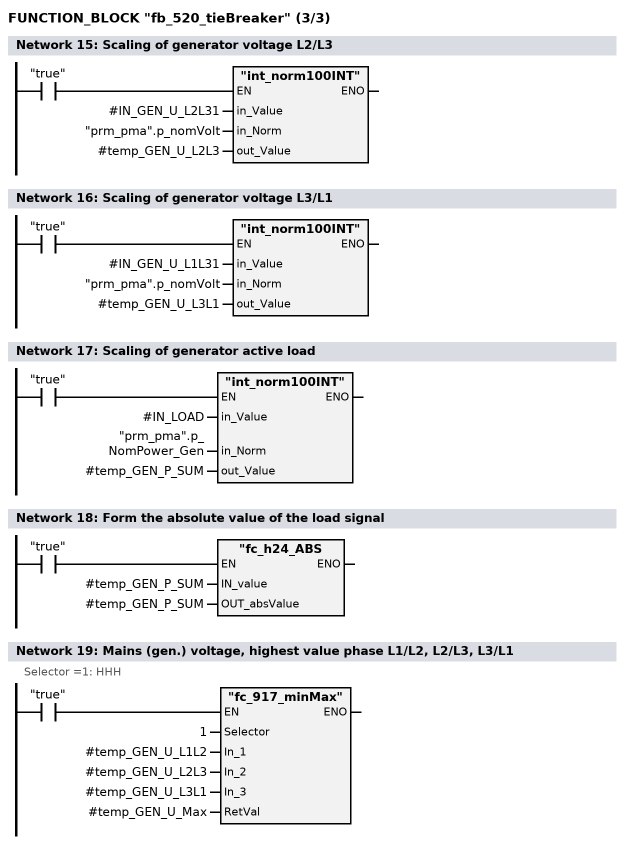
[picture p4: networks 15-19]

      U     "true";
      SPBNB _00b;
      CALL "int_norm100INT" (
           in_Value                 := #IN_GEN_U_L2L31,
           in_Norm                  := "prm_pma".p_nomVolt,
           out_Value                := #temp_GEN_U_L2L3);
_00b: NOP   0;
NETWORK
TITLE =Scaling of generator voltage L3/L1

      U     "true";
      SPBNB _00c;
      CALL "int_norm100INT" (
           in_Value                 := #IN_GEN_U_L1L31,
           in_Norm                  := "prm_pma".p_nomVolt,
           out_Value                := #temp_GEN_U_L3L1);
_00c: NOP   0;
NETWORK
TITLE =Scaling of generator active load

      U     "true";
      SPBNB _00d;
      CALL "int_norm100INT" (
           in_Value                 := #IN_LOAD,
           in_Norm                  := "prm_pma".p_NomPower_Gen,
           out_Value                := #temp_GEN_P_SUM);
_00d: NOP   0;
NETWORK
TITLE =Form the absolute value of the load signal

      U     "true";
      SPBNB _00e;
      CALL "fc_h24_ABS(INT)" (
           IN_value                 := #temp_GEN_P_SUM,
           OUT_absValue             := #temp_GEN_P_SUM);
_00e: NOP   0;
NETWORK
TITLE =Mains (gen.) voltage, highest value phase L1/L2, L2/L3, L3/L1
//Selector =1: HHH
      U     "true";
      SPBNB _00f;
      CALL "fc_917_minMax" (
           Selector                 := 1,
           In_1                     := #temp_GEN_U_L1L2,
           In_2                     := #temp_GEN_U_L2L3,
           In_3                     := #temp_GEN_U_L3L1,
           RetVal                   := #temp_GEN_U_Max);
_00f: NOP   0;
NETWORK
TITLE =Blackout monitoring
//For the blackout monitoring three signals are combined: The signals "Blackout"
//and not "Busbar voltage present" from the contactors for busbar monitoring and
//the actual value of voltage from the converter, which has to be below a certain
//limit.
      U     #IN_blackout_bus;
      UN    #IN_VoltAvail_bus;
      U(    ;
      L     #temp_GEN_U_Max;
      L     "prm_pma".p_Vblackout;
      <I    ;
      )     ;
      =     L     48.0;
      U     L     48.0;
      L     "prm_pma".p_Tblackout;
      SE    "dlyT_BlackBus_Tiebrk";
      NOP   0;
      NOP   0;
      LC    "dlyT_BlackBus_Tiebrk";
      T     #temp_RdlyTrun_blackBus;
      U     "dlyT_BlackBus_Tiebrk";
      =     #temp_blackBus;
      U     L     48.0;
      BLD   102;
      =     #temp_blackout_undly;
NETWORK
TITLE =Blackout detecting time is running

      U     #temp_blackout_undly;
      UN    #temp_blackBus;
      =     #temp_blackoutT_run;
NETWORK
TITLE =Indication "Failure busbar/blackout monitoring"
//If both signals "Blackout" and "Busbar voltage present" from the contactors for
//busbar monitoring are present or both are not present, there is a failure in
//the
//busbar monitoring.
      U     #IN_reset;
      R     #OUT_e_busbar_monit;
      U(    ;
      U(    ;
      U     #IN_blackout_bus;
      U     #IN_VoltAvail_bus;
      O     ;
      UN    #IN_blackout_bus;
      UN    #IN_VoltAvail_bus;
      )     ;
      L     "prm_pma".p_TFBusbar;
      SE    "dlyT_BusbarFail_TieBrk";
      NOP   0;
      NOP   0;
      NOP   0;
      U     "dlyT_BusbarFail_TieBrk";
      )     ;
      S     #OUT_e_busbar_monit;
      NOP   0;
NETWORK
TITLE =Generator protection (FB56)
//In this case: Generator means busbar, busbar means transferline!
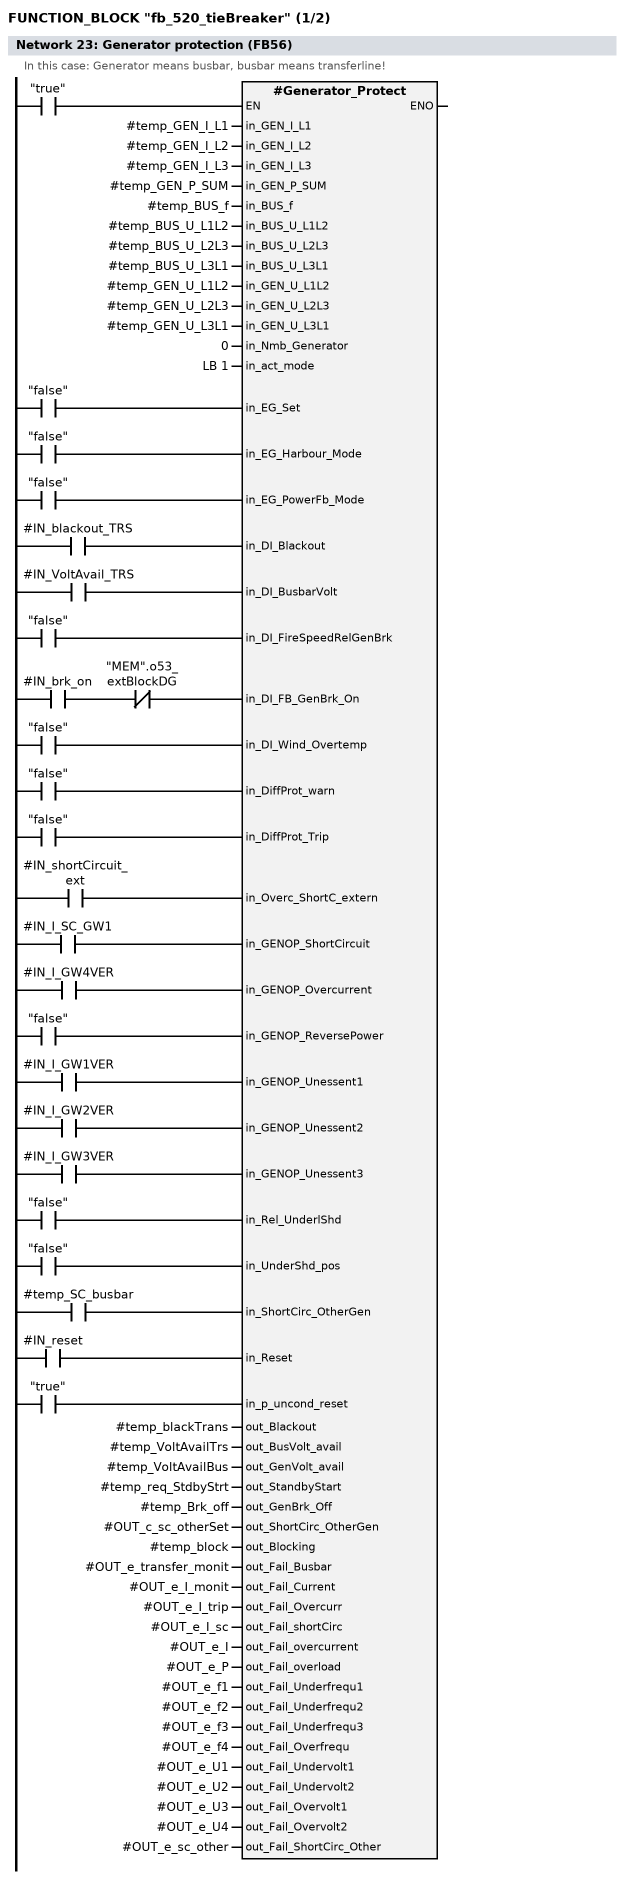
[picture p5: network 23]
      U     "false";
      =     L     48.0;
      BLD   103;
      U     "false";
      =     L     48.1;
      BLD   103;
      U     "false";
      =     L     48.2;
      BLD   103;
      U     #IN_blackout_TRS;
      =     L     48.3;
      BLD   103;
      U     #IN_VoltAvail_TRS;
      =     L     48.4;
      BLD   103;
      U     "false";
      =     L     48.5;
      BLD   103;
      U     #IN_brk_on;
      UN    "MEM".o53_extBlockDG;
      =     L     48.6;
      BLD   103;
      U     "false";
      =     L     48.7;
      BLD   103;
      U     "false";
      =     L     49.0;
      BLD   103;
      U     "false";
      =     L     49.1;
      BLD   103;
      U     #IN_shortCircuit_ext;
      =     L     49.2;
      BLD   103;
      U     #IN_I_SC_GW1;
      =     L     49.3;
      BLD   103;
      U     #IN_I_GW4VER;
      =     L     49.4;
      BLD   103;
      U     "false";
      =     L     49.5;
      BLD   103;
      U     #IN_I_GW1VER;
      =     L     49.6;
      BLD   103;
      U     #IN_I_GW2VER;
      =     L     49.7;
      BLD   103;
      U     #IN_I_GW3VER;
      =     L     50.0;
      BLD   103;
      U     "false";
      =     L     50.1;
      BLD   103;
      U     "false";
      =     L     50.2;
      BLD   103;
      U     #temp_SC_busbar;
      =     L     50.3;
      BLD   103;
      U     #IN_reset;
      =     L     50.4;
      BLD   103;
      U     "true";
      =     L     50.5;
      BLD   103;
      U     "true";
      SPBNB _010;
      CALL #Generator_Protect (
           in_GEN_I_L1              := #temp_GEN_I_L1,
           in_GEN_I_L2              := #temp_GEN_I_L2,
           in_GEN_I_L3              := #temp_GEN_I_L3,
           in_GEN_P_SUM             := #temp_GEN_P_SUM,
           in_BUS_f                 := #temp_BUS_f,
           in_BUS_U_L1L2            := #temp_BUS_U_L1L2,
           in_BUS_U_L2L3            := #temp_BUS_U_L2L3,
           in_BUS_U_L3L1            := #temp_BUS_U_L3L1,
           in_GEN_U_L1L2            := #temp_GEN_U_L1L2,
           in_GEN_U_L2L3            := #temp_GEN_U_L2L3,
           in_GEN_U_L3L1            := #temp_GEN_U_L3L1,
           in_Nmb_Generator         := 0,
           in_act_mode              := LB     1,
           in_EG_Set                := L     48.0,
           in_EG_Harbour_Mode       := L     48.1,
           in_EG_PowerFb_Mode       := L     48.2,
           in_DI_Blackout           := L     48.3,
           in_DI_BusbarVolt         := L     48.4,
           in_DI_FireSpeedRelGenBrk := L     48.5,
           in_DI_FB_GenBrk_On       := L     48.6,
           in_DI_Wind_Overtemp      := L     48.7,
           in_DiffProt_warn         := L     49.0,
           in_DiffProt_Trip         := L     49.1,
           in_Overc_ShortC_extern   := L     49.2,
           in_GENOP_ShortCircuit    := L     49.3,
           in_GENOP_Overcurrent     := L     49.4,
           in_GENOP_ReversePower    := L     49.5,
           in_GENOP_Unessent1       := L     49.6,
           in_GENOP_Unessent2       := L     49.7,
           in_GENOP_Unessent3       := L     50.0,
           in_Rel_UnderlShd         := L     50.1,
           in_UnderShd_pos          := L     50.2,
           in_ShortCirc_OtherGen    := L     50.3,
           in_Reset                 := L     50.4,
           in_p_uncond_reset        := L     50.5,
           out_Blackout             := #temp_blackTrans,
           out_BusVolt_avail        := #temp_VoltAvailTrs,
           out_GenVolt_avail        := #temp_VoltAvailBus,
           out_StandbyStart         := #temp_req_StdbyStrt,
           out_GenBrk_Off           := #temp_Brk_off,
           out_ShortCirc_OtherGen   := #OUT_c_sc_otherSet,
           out_Blocking             := #temp_block,
           out_Fail_Busbar          := #OUT_e_transfer_monit,
           out_Fail_Current         := #OUT_e_I_monit,
           out_Fail_Overcurr        := #OUT_e_I_trip,
           out_Fail_shortCirc       := #OUT_e_I_sc,
           out_Fail_overcurrent     := #OUT_e_I,
           out_Fail_overload        := #OUT_e_P,
           out_Fail_Underfrequ1     := #OUT_e_f1,
           out_Fail_Underfrequ2     := #OUT_e_f2,
           out_Fail_Underfrequ3     := #OUT_e_f3,
           out_Fail_Overfrequ       := #OUT_e_f4,
           out_Fail_Undervolt1      := #OUT_e_U1,
           out_Fail_Undervolt2      := #OUT_e_U2,
           out_Fail_Overvolt1       := #OUT_e_U3,
           out_Fail_Overvolt2       := #OUT_e_U4,
           out_Fail_ShortCirc_Other := #OUT_e_sc_other);


_010: NOP   0;
NETWORK
TITLE =Indication "blackout busbar"
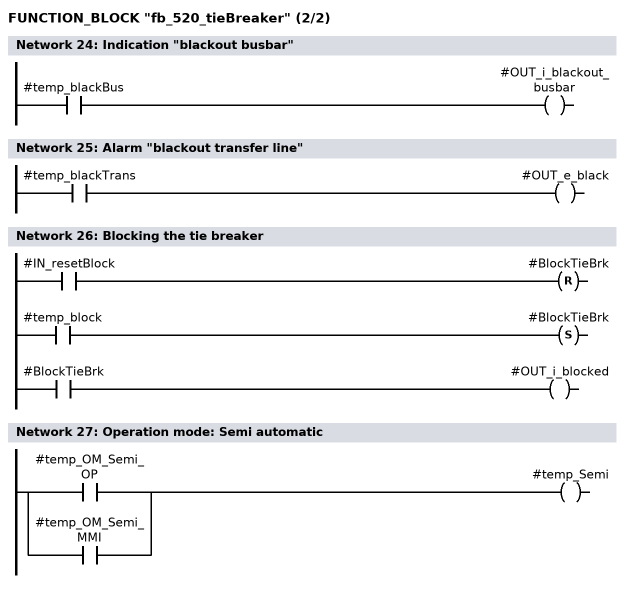
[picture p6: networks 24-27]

      U     #temp_blackBus;
      =     #OUT_i_blackout_busbar;
NETWORK
TITLE =Alarm "blackout transfer line"

      U     #temp_blackTrans;
      =     #OUT_e_black;
NETWORK
TITLE =Blocking the tie breaker

      U     #IN_resetBlock;
      R     #BlockTieBrk;
      U     #temp_block;
      S     #BlockTieBrk;
      U     #BlockTieBrk;
      =     #OUT_i_blocked;
NETWORK
TITLE =Operation mode: Semi automatic

      O     #temp_OM_Semi_OP;
      O     #temp_OM_Semi_MMI;
      =     #temp_Semi;
NETWORK
TITLE =Blackout on busbar or transferline

      X     #temp_blackBus;
      X     #temp_blackTrans;
      =     #temp_blackout;
NETWORK
TITLE =Voltage busbar or transferline available

      X     #temp_VoltAvailTrs;
      X     #temp_VoltAvailBus;
      =     #temp_voltAvailPrtct;
NETWORK
TITLE =Blackout on busbar and transferline
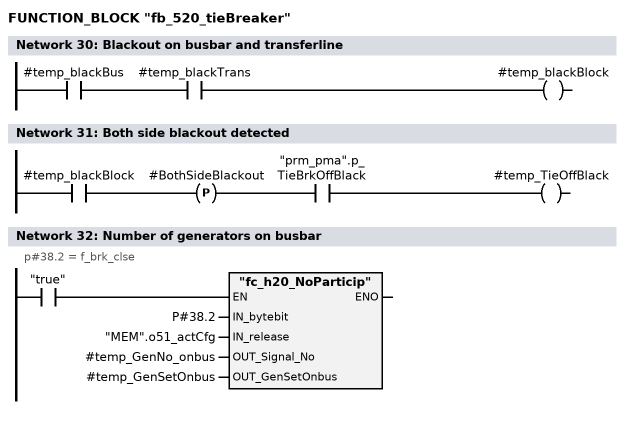
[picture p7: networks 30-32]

      U     #temp_blackBus;
      U     #temp_blackTrans;
      =     #temp_blackBlock;
NETWORK
TITLE =Both side blackout detected

      U     #temp_blackBlock;
      FP    #BothSideBlackout;
      U     "prm_pma".p_TieBrkOffBlack;
      =     #temp_TieOffBlack;
NETWORK
TITLE =Number of generators on busbar
//p#38.2 = f_brk_clse
      U     "true";
      SPBNB _011;
      CALL "fc_h20_NoParticip" (
           IN_bytebit               := P#38.2,
           IN_release               := "MEM".o51_actCfg,
           OUT_Signal_No            := #temp_GenNo_onbus,
           OUT_GenSetOnbus          := #temp_GenSetOnbus);
_011: NOP   0;
NETWORK
TITLE =Determine new generator on busbar
//Check whether the new generator on busbar is a generator of the own busbar
      L     #memo_GenSetOnBus;
      L     #temp_GenSetOnbus;
      ==I   ;
      SPB   actG;
      XOW   ;
      L     #temp_GenSetOnbus;
      UW    ;
      T     #memo_newGenSet;
      L     #temp_GenSetOnbus;
      T     #memo_GenSetOnBus;

actG: L     #memo_newGenSet;
      L     #temp_CfgBusbar;
      UW    ;
      L     0;
      <>I   ;
      =     #temp_GenSetOwn;

NETWORK
TITLE =Number of allowed generators on busbar exceeded
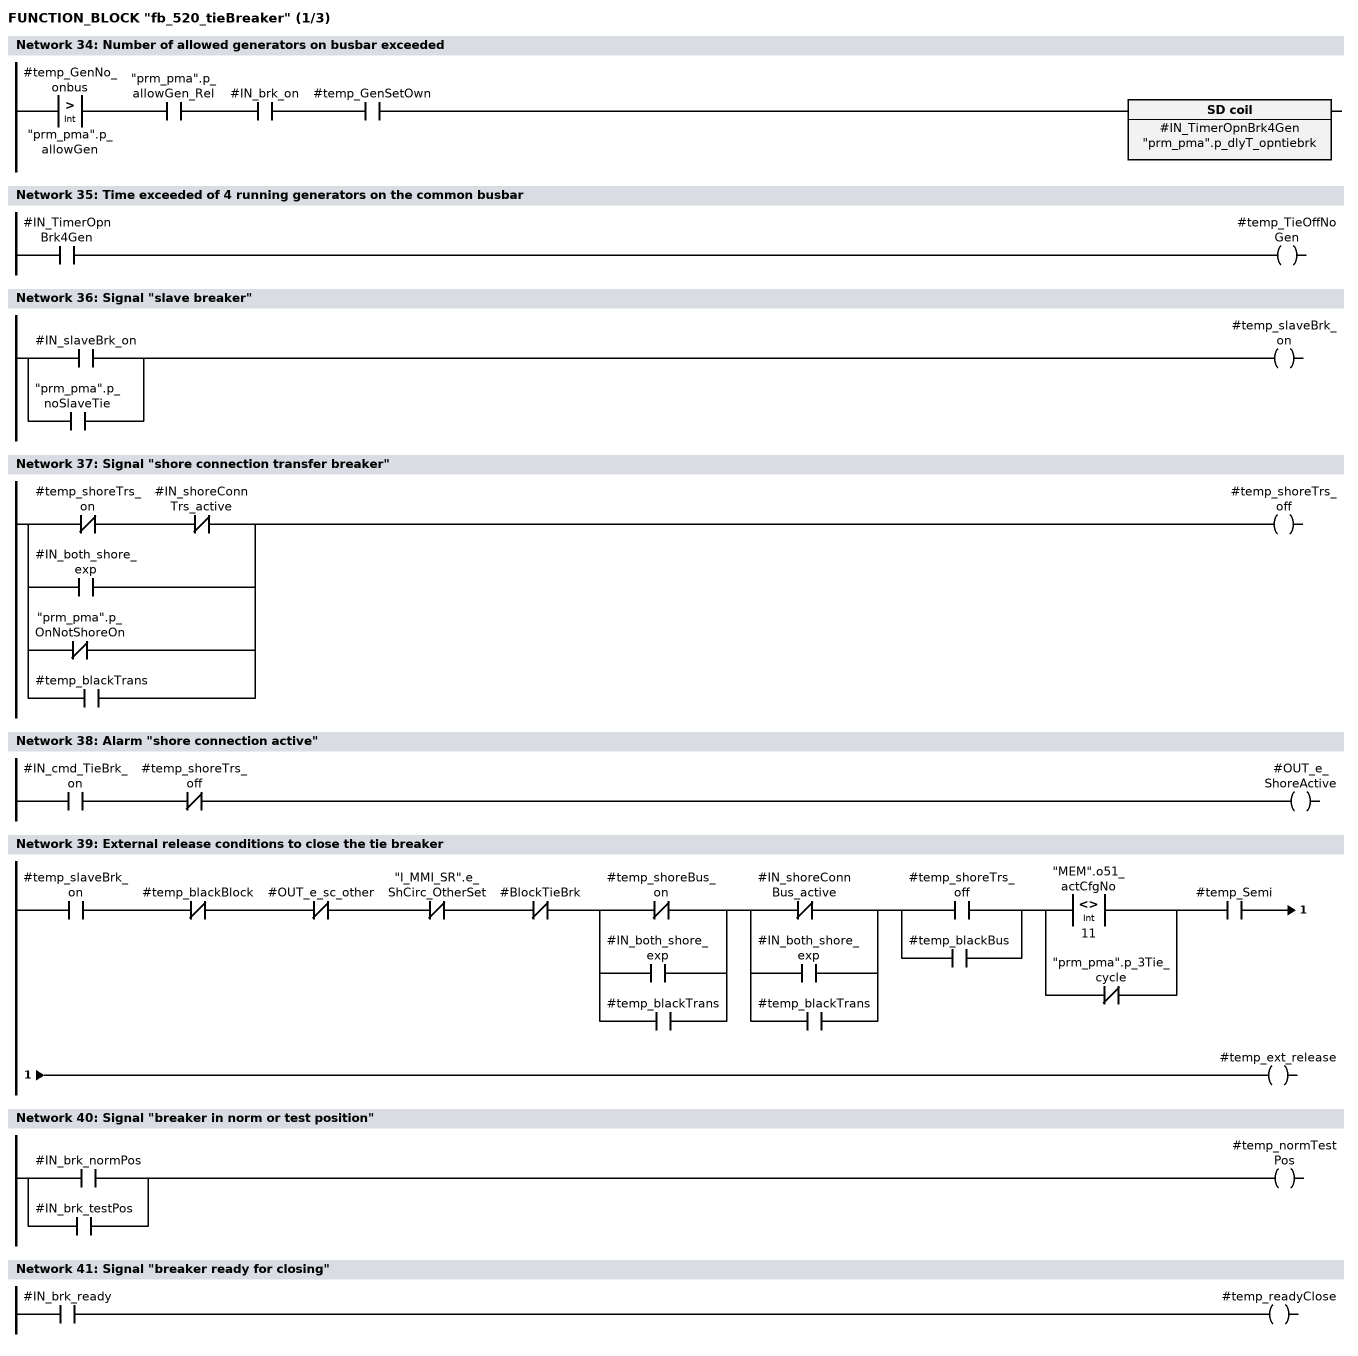
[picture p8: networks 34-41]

      U(    ;
      L     #temp_GenNo_onbus;
      L     "prm_pma".p_allowGen;
      >I    ;
      )     ;
      U     "prm_pma".p_allowGen_Rel;
      U     #IN_brk_on;
      U     #temp_GenSetOwn;
      L     "prm_pma".p_dlyT_opntiebrk;
      SE    #IN_TimerOpnBrk4Gen;
NETWORK
TITLE =Time exceeded of 4 running generators on the common busbar

      U     #IN_TimerOpnBrk4Gen;
      =     #temp_TieOffNoGen;
NETWORK
TITLE =Signal "slave breaker"

      O     #IN_slaveBrk_on;
      O     "prm_pma".p_noSlaveTie;
      =     #temp_slaveBrk_on;
NETWORK
TITLE =Signal "shore connection transfer breaker"

      UN    #temp_shoreTrs_on;
      UN    #IN_shoreConnTrs_active;
      O     #IN_both_shore_exp;
      ON    "prm_pma".p_OnNotShoreOn;
      O     #temp_blackTrans;
      =     #temp_shoreTrs_off;
NETWORK
TITLE =Alarm "shore connection active"

      U     #IN_cmd_TieBrk_on;
      UN    #temp_shoreTrs_off;
      =     #OUT_e_ShoreActive;
NETWORK
TITLE =External release conditions to close the tie breaker

      U     #temp_slaveBrk_on;
      UN    #temp_blackBlock;
      UN    #OUT_e_sc_other;
      UN    "I_MMI_SR".e_ShCirc_OtherSet;
      UN    #BlockTieBrk;
      U(    ;
      ON    #temp_shoreBus_on;
      O     #IN_both_shore_exp;
      O     #temp_blackTrans;
      )     ;
      U(    ;
      ON    #IN_shoreConnBus_active;
      O     #IN_both_shore_exp;
      O     #temp_blackTrans;
      )     ;
      U(    ;
      O     #temp_shoreTrs_off;
      O     #temp_blackBus;
      )     ;
      U(    ;
      O(    ;
      L     "MEM".o51_actCfgNo;
      L     11;
      <>I   ;
      )     ;
      ON    "prm_pma".p_3Tie_cycle;
      )     ;
      U     #temp_Semi;
      =     #temp_ext_release;
NETWORK
TITLE =Signal "breaker in norm or test position"

      O     #IN_brk_normPos;
      O     #IN_brk_testPos;
      =     #temp_normTestPos;
NETWORK
TITLE =Signal "breaker ready for closing"

      U     #IN_brk_ready;
      =     #temp_readyClose;
NETWORK
TITLE =Control of tie breaker (FB51)
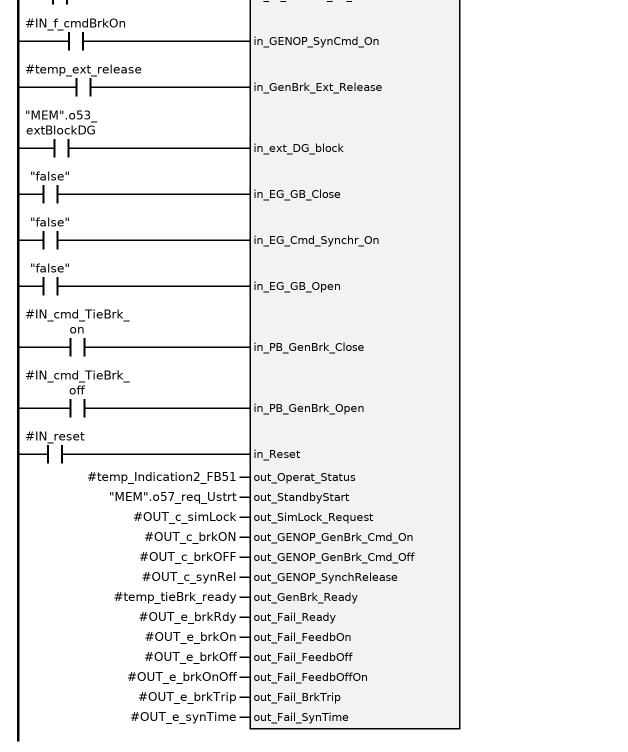
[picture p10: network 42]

      U     "false";
      =     L     48.0;
      BLD   103;
      U     "false";
      =     L     48.1;
      BLD   103;
      U     #temp_blackout;
      =     L     48.2;
      BLD   103;
      U     #IN_simLock_blc;
      =     L     48.3;
      BLD   103;
      U     #IN_simLock_err;
      =     L     48.4;
      BLD   103;
      U     #IN_simLockRel;
      =     L     48.5;
      BLD   103;
      U     "true";
      =     L     48.6;
      BLD   103;
      U     "false";
      =     L     48.7;
      BLD   103;
      U     "false";
      =     L     49.0;
      BLD   103;
      U(    ;
      O     #temp_TieOffBlack;
      O     #temp_TieOffNoGen;
      O     #temp_SC_busbar;
      O     #OUT_c_sc_otherSet;
      ON    #IN_PB_TieBrk_off;
      O(    ;
      U     #temp_slaveBrk_on;
      FN    #pulse_SlvBrk;
      )     ;
      )     ;
      =     L     49.1;
      BLD   103;
      U     #temp_Brk_off;
      =     L     49.2;
      BLD   103;
      U     "false";
      =     L     49.3;
      BLD   103;
      U     "false";
      =     L     49.4;
      BLD   103;
      U     "true";
      =     L     49.5;
      BLD   103;
      U     #IN_brk_ready;
      =     L     49.6;
      BLD   103;
      U     "false";
      =     L     49.7;
      BLD   103;
      U     #IN_brk_normPos;
      UN    "MEM".o57_extBlock;
      =     L     50.0;
      BLD   103;
      U     #IN_brk_testPos;
      UN    "MEM".o57_extBlock;
      =     L     50.1;
      BLD   103;
      U     #IN_brk_on;
      =     L     50.2;
      BLD   103;
      U     #IN_brk_off;
      =     L     50.3;
      BLD   103;
      U     #IN_f_cmdBrkOn;
      =     L     50.4;
      BLD   103;
      U     #temp_ext_release;
      =     L     50.5;
      BLD   103;
      U     "MEM".o53_extBlockDG;
      =     L     50.6;
      BLD   103;
      U     "false";
      =     L     50.7;
      BLD   103;
      U     "false";
      =     L     51.0;
      BLD   103;
      U     "false";
      =     L     51.1;
      BLD   103;
      U     #IN_cmd_TieBrk_on;
      =     L     51.2;
      BLD   103;
      U     #IN_cmd_TieBrk_off;
      =     L     51.3;
      BLD   103;
      U     #IN_reset;
      =     L     51.6;
      BLD   103;
      U     "true";
      SPBNB _012;
      CALL #Breaker_control (
           in_DGLoad_off            := L     48.0,
           in_Nmb_Gen_LoadSh        := 0,
           in_act_mode              := #IN_mode,
           in_EG_Set                := L     48.1,
           in_Blackout              := L     48.2,
           in_SimLock_Blocked       := L     48.3,
           in_SimLock_Fault         := L     48.4,
           in_SimLock_Release       := L     48.5,
           in_DGWG_run              := L     48.6,
           in_DGWG_Stop             := L     48.7,
           in_GenBrkOff_LoadRed     := L     49.0,
           in_DGWG_GenBrk_Cmd_Off   := L     49.1,
           in_DGWG_GenBrk_Cmd_Trip  := L     49.2,
           in_ChOver_Blackout       := L     49.3,
           in_Standby_ReadyConn     := L     49.4,
           in_ShoreConn_Off         := L     49.5,
           in_DI_GenBrk_ReadyClose  := L     49.6,
           in_DI_GenBrk_Tripped     := L     49.7,
           in_DI_GenBrk_PosNorm     := L     50.0,
           in_DI_GenBrk_PosTest     := L     50.1,
           in_DI_GenBrk_FB_On       := L     50.2,
           in_DI_GenBrk_FB_Off      := L     50.3,
           in_GENOP_SynCmd_On       := L     50.4,
           in_GenBrk_Ext_Release    := L     50.5,
           in_ext_DG_block          := L     50.6,
           in_EG_GB_Close           := L     50.7,
           in_EG_Cmd_Synchr_On      := L     51.0,
           in_EG_GB_Open            := L     51.1,
           in_PB_GenBrk_Close       := L     51.2,
           in_PB_GenBrk_Open        := L     51.3,
           in_Reset                 := L     51.6,
           out_Operat_Status        := #temp_Indication2_FB51,
           out_StandbyStart         := "MEM".o57_req_Ustrt,
           out_SimLock_Request      := #OUT_c_simLock,
           out_GENOP_GenBrk_Cmd_On  := #OUT_c_brkON,
           out_GENOP_GenBrk_Cmd_Off := #OUT_c_brkOFF,
           out_GENOP_SynchRelease   := #OUT_c_synRel,
           out_GenBrk_Ready         := #temp_tieBrk_ready,
           out_Fail_Ready           := #OUT_e_brkRdy,
           out_Fail_FeedbOn         := #OUT_e_brkOn,
           out_Fail_FeedbOff        := #OUT_e_brkOff,
           out_Fail_FeedbOffOn      := #OUT_e_brkOnOff,
           out_Fail_BrkTrip         := #OUT_e_brkTrip,
           out_Fail_SynTime         := #OUT_e_synTime);

_012: NOP   0;
NETWORK
TITLE =As long as the closing process is running lock the controller
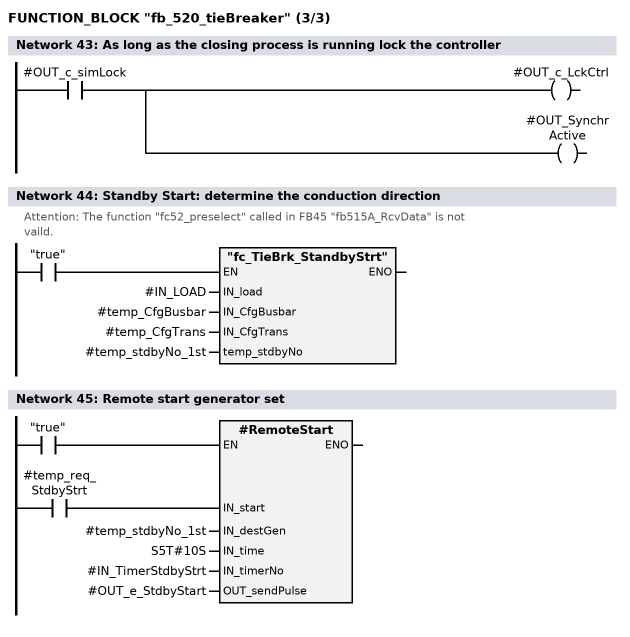
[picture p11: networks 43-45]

      U     #OUT_c_simLock;
      =     #OUT_c_LckCtrl;
      =     #OUT_SynchrActive;
NETWORK
TITLE =Standby Start: determine the conduction direction
//Attention: The function "fc52_preselect" called in FB45 "fb515A_RcvData" is not
//           vaild.
      U     "true";
      SPBNB _013;
      CALL "fc_TieBrk_StandbyStrt" (
           IN_load                  := #IN_LOAD,
           IN_CfgBusbar             := #temp_CfgBusbar,
           IN_CfgTrans              := #temp_CfgTrans,
           temp_stdbyNo             := #temp_stdbyNo_1st);
_013: NOP   0;
NETWORK
TITLE =Remote start generator set

      U     #temp_req_StdbyStrt;
      =     L     48.0;
      BLD   103;
      U     "true";
      SPBNB _014;
      CALL #RemoteStart (
           IN_start                 := L     48.0,
           IN_destGen               := #temp_stdbyNo_1st,
           IN_time                  := S5T#10S,
           IN_timerNo               := #IN_TimerStdbyStrt,
           OUT_sendPulse            := #OUT_e_StdbyStart);
_014: NOP   0;
NETWORK
TITLE =Indication line1:No.37: "Tie breaker closed" without kW display

      L     37;
      U     #IN_brk_on;
      U     #temp_blackout;
      SPB   idOP;
NETWORK
TITLE =Indication line1:No.38: "Tie breaker closed" with kW display

      L     38;
      U     #IN_brk_on;
      UN    #temp_blackout;
      SPB   idOP;
NETWORK
TITLE =Indication line1:No.30: "_______" (No indication)
//If there is no indication coming from this FB, "30" is delivered.
      L     30;
idOP: T     #temp_Operat_Status;
NETWORK
TITLE =Indication line 2, no. 1: "press confirmation"

      L     1;
      U     #IN_pressCnfrm;
      SPB   indi;
NETWORK
TITLE =Indication line 2, no. 20: "Blocked"

      L     20;
      U     #BlockTieBrk;
      SPB   indi;
NETWORK
TITLE =Indication line 2, no. 12: "Tie breaker ready"

      L     12;
      U     #temp_ext_release;
      U     #temp_tieBrk_ready;
      U     #temp_Semi;
      UN    #IN_brk_on;
      UN    #BlockTieBrk;
      UN    #IN_simLock_err;
      SPB   indi;

NETWORK
TITLE =Indication line 2, no. 11: "Tie breaker not ready"

      L     11;
      U(    ;
      ON    #temp_ext_release;
      ON    #temp_tieBrk_ready;
      ON    #temp_Semi;
      O     #BlockTieBrk;
      O     #IN_simLock_err;
      )     ;
      UN    #IN_brk_on;
      SPB   indi;
NETWORK
TITLE =Indication line 2, no. 10: "_______" (No indication)
//If there is no indication coming for this line, "10" is delivered.
      L     10;
indi: T     #out_ind_line2_var;
NETWORK
TITLE =Transfer of indication line 1, no. 41,44,45 (FB51-->DB101)
//During load reduction FB51 will output number "41". This number is transfered
//to OP/MMI and the transfer of the indication number from FB47 is suppressed.
//The
//other time FB51 will output number "30" and the number from FB47 is transfered
//to OP/MMI.
      L     30;
      L     #temp_Indication2_FB51;
      <>I   ;
      SPB   ind;
NETWORK
TITLE =Transfer of indication no., line 2 (FB47-->DB101)

      L     #temp_Operat_Status;
ind:  T     #OUT_ind_line1_stat;
NETWORK
TITLE =Indication "ready breaker "

      L     LB     4;
      T     #OUT_ind_ready;

END_FUNCTION_BLOCK

DATA_BLOCK "tieB_1"
TITLE =
VERSION : 0.0

"fb_520_tieBreaker"
BEGIN
   IN_synchrToOwnBus := FALSE;
   IN_cmd_TieBrk_on := FALSE;
   IN_cmd_TieBrk_off := FALSE;
   IN_PB_TieBrk_off := FALSE;
   IN_blackout_bus := FALSE;
   IN_VoltAvail_bus := FALSE;
   IN_blackout_TRS := FALSE;
   IN_VoltAvail_TRS := FALSE;
   IN_slaveBrk_on := FALSE;
   IN_shoreConnBus_active := FALSE;
   IN_shoreConnTrs_active := FALSE;
   IN_both_shore_exp := FALSE;
   IN_shortCircuit_otherG := FALSE;
   IN_shortCircuit_ext := FALSE;
   IN_GEN_I_L1 := 0;
   IN_GEN_I_L2 := 0;
   IN_GEN_I_L3 := 0;
   IN_LOAD := 0;
   IN_BUS_f := 0;
   IN_GEN_f := 0;
   IN_BUS_U_L1L2 := 0;
   IN_BUS_U_L2L3 := 0;
   IN_BUS_U_L1L3 := 0;
   IN_GEN_U_L1L21 := 0;
   IN_GEN_U_L2L31 := 0;
   IN_GEN_U_L1L31 := 0;
   IN_I_SC_GW1 := FALSE;
   IN_I_GW1VER := FALSE;
   IN_I_GW2VER := FALSE;
   IN_I_GW3VER := FALSE;
   IN_I_GW4VER := FALSE;
   IN_simLock_blc := FALSE;
   IN_simLock_err := FALSE;
   IN_simLockRel := FALSE;
   IN_brk_ready := FALSE;
   IN_brk_normPos := FALSE;
   IN_brk_testPos := FALSE;
   IN_brk_on := FALSE;
   IN_brk_off := FALSE;
   IN_othBrk_on := FALSE;
   IN_f_cmdBrkOn := FALSE;
   IN_reset := FALSE;
   IN_resetBlock := FALSE;
   IN_pressCnfrm := FALSE;
   IN_mode := B#16#0;
   IN_TimerStdbyStrt := T 0;
   IN_TimerOpnBrk4Gen := T 0;
   OUT_SynchrActive := FALSE;
   OUT_c_LckCtrl := FALSE;
   OUT_c_simLock := FALSE;
   OUT_c_brkON := FALSE;
   OUT_c_brkOFF := FALSE;
   OUT_c_synRel := FALSE;
   OUT_c_reqStrt := FALSE;
   OUT_c_sc_otherSet := FALSE;
   OUT_i_blocked := FALSE;
   OUT_i_blackout_busbar := FALSE;
   OUT_i_blackout_trans := FALSE;
   OUT_i_CfgBusbar := 0;
   OUT_e_transfer_monit := FALSE;
   OUT_e_busbar_monit := FALSE;
   OUT_e_I_monit := FALSE;
   OUT_e_I_trip := FALSE;
   OUT_e_I := FALSE;
   OUT_e_P := FALSE;
   OUT_e_f1 := FALSE;
   OUT_e_f2 := FALSE;
   OUT_e_f3 := FALSE;
   OUT_e_f4 := FALSE;
   OUT_e_U1 := FALSE;
   OUT_e_U2 := FALSE;
   OUT_e_U3 := FALSE;
   OUT_e_U4 := FALSE;
   OUT_e_I_sc := FALSE;
   OUT_e_sc_other := FALSE;
   OUT_e_black := FALSE;
   OUT_e_brkRdy := FALSE;
   OUT_e_brkOn := FALSE;
   OUT_e_brkOff := FALSE;
   OUT_e_brkOnOff := FALSE;
   OUT_e_brkTrip := FALSE;
   OUT_e_synTime := FALSE;
   OUT_e_StdbyStart := FALSE;
   OUT_e_ShoreActive := FALSE;
   OUT_ind_ready := B#16#0;
   OUT_ind_line1_stat := 0;
   out_ind_line2_var := 0;
   Gen_Protect.in_GEN_I_L1 := 0;
   Gen_Protect.in_GEN_I_L2 := 0;
   Gen_Protect.in_GEN_I_L3 := 0;
   Gen_Protect.in_GEN_P_SUM := 0;
   Gen_Protect.in_BUS_f := 0;
   Gen_Protect.in_BUS_U_L1L2 := 0;
   Gen_Protect.in_BUS_U_L2L3 := 0;
   Gen_Protect.in_BUS_U_L3L1 := 0;
   Gen_Protect.in_GEN_U_L1L2 := 0;
   Gen_Protect.in_GEN_U_L2L3 := 0;
   Gen_Protect.in_GEN_U_L3L1 := 0;
   Gen_Protect.in_Nmb_Generator := 0;
   Gen_Protect.in_act_mode := B#16#0;
   Gen_Protect.in_EG_Set := FALSE;
   Gen_Protect.in_EG_Harbour_Mode := FALSE;
   Gen_Protect.in_EG_PowerFb_Mode := FALSE;
   Gen_Protect.in_DI_Blackout := FALSE;
   Gen_Protect.in_DI_BusbarVolt := FALSE;
   Gen_Protect.in_DI_FireSpeedRelGenBrk := FALSE;
   Gen_Protect.in_DI_FB_GenBrk_On := FALSE;
   Gen_Protect.in_DI_Wind_Overtemp := FALSE;
   Gen_Protect.in_DiffProt_warn := FALSE;
   Gen_Protect.in_DiffProt_Trip := FALSE;
   Gen_Protect.in_Overc_ShortC_extern := FALSE;
   Gen_Protect.in_GENOP_ShortCircuit := FALSE;
   Gen_Protect.in_GENOP_Overcurrent := FALSE;
   Gen_Protect.in_GENOP_ReversePower := FALSE;
   Gen_Protect.in_GENOP_Unessent1 := FALSE;
   Gen_Protect.in_GENOP_Unessent2 := FALSE;
   Gen_Protect.in_GENOP_Unessent3 := FALSE;
   Gen_Protect.in_Rel_UnderlShd := FALSE;
   Gen_Protect.in_UnderShd_pos := FALSE;
   Gen_Protect.in_ShortCirc_OtherGen := FALSE;
   Gen_Protect.in_Reset := FALSE;
   Gen_Protect.in_p_uncond_reset := FALSE;
   Gen_Protect.out_Blackout := FALSE;
   Gen_Protect.out_BusVolt_avail := FALSE;
   Gen_Protect.out_GenVolt_avail := FALSE;
   Gen_Protect.out_StandbyStart := FALSE;
   Gen_Protect.out_Uness1_Off := FALSE;
   Gen_Protect.out_Uness2_Off := FALSE;
   Gen_Protect.out_Uness3_Off := FALSE;
   Gen_Protect.out_GenBrk_Off := FALSE;
   Gen_Protect.out_ShortCirc_OtherGen := FALSE;
   Gen_Protect.out_VoltContr_Off := FALSE;
   Gen_Protect.out_UndelayStop := FALSE;
   Gen_Protect.out_Blocking := FALSE;
   Gen_Protect.out_ChOver_Semi := FALSE;
   Gen_Protect.out_ChOver_Blackout := FALSE;
   Gen_Protect.out_Underload_Limit := FALSE;
   Gen_Protect.out_Underload_Shd := FALSE;
   Gen_Protect.out_Fail_Busbar := FALSE;
   Gen_Protect.out_Fail_Current := FALSE;
   Gen_Protect.out_Fail_Overcurr := FALSE;
   Gen_Protect.out_Fail_shortCirc := FALSE;
   Gen_Protect.out_Fail_RevPower := FALSE;
   Gen_Protect.out_Fail_overcurrent := FALSE;
   Gen_Protect.out_Fail_overload := FALSE;
   Gen_Protect.out_Fail_Underfrequ1 := FALSE;
   Gen_Protect.out_Fail_Underfrequ2 := FALSE;
   Gen_Protect.out_Fail_Underfrequ3 := FALSE;
   Gen_Protect.out_Fail_Overfrequ := FALSE;
   Gen_Protect.out_Fail_Undervolt1 := FALSE;
   Gen_Protect.out_Fail_Undervolt2 := FALSE;
   Gen_Protect.out_Fail_Overvolt1 := FALSE;
   Gen_Protect.out_Fail_Overvolt2 := FALSE;
   Gen_Protect.out_Fail_ShortCirc_Other := FALSE;
   Gen_Protect.out_Fail_DiffProt_Warn := FALSE;
   Gen_Protect.out_Fail_DiffProt_Trip := FALSE;
   Gen_Protect.out_Fail_Wind_Overtemp := FALSE;
   Gen_Protect.out_Fail_Underload := FALSE;
   Gen_Protect.out_Fail_Underl_SD := FALSE;
   Gen_Protect.out_Spare_1 := FALSE;
   Gen_Protect.out_Spare_2 := FALSE;
   Gen_Protect.out_PrtcEG_sign := DW#16#0;
   Gen_Protect.stat_GEN_I_Min := 0;
   Gen_Protect.stat_GEN_I_Max := 0;
   Gen_Protect.stat_GEN_I_Mean := 0;
   Gen_Protect.stat_BUS_U_Min := 0;
   Gen_Protect.stat_BUS_U_Max := 0;
   Gen_Protect.stat_GEN_U_Min := 0;
   Gen_Protect.stat_GEN_U_Max := 0;
   Gen_Protect.stat_Limit_I1 := FALSE;
   Gen_Protect.stat_Limit_I2 := FALSE;
   Gen_Protect.stat_Limit_I3 := FALSE;
   Gen_Protect.stat_Limit_I4 := FALSE;
   Gen_Protect.stat_Limit_I5 := FALSE;
   Gen_Protect.stat_Limit_I6 := FALSE;
   Gen_Protect.stat_Limit_I7 := FALSE;
   Gen_Protect.stat_Limit_P1 := FALSE;
   Gen_Protect.stat_Limit_P2 := FALSE;
   Gen_Protect.stat_Limit_P3 := FALSE;
   Gen_Protect.stat_Limit_P4 := FALSE;
   Gen_Protect.stat_Limit_P5 := FALSE;
   Gen_Protect.stat_Limit_P6 := FALSE;
   Gen_Protect.stat_Limit_P7 := FALSE;
   Gen_Protect.stat_Limit_f1 := FALSE;
   Gen_Protect.stat_Limit_f2 := FALSE;
   Gen_Protect.stat_Limit_f3 := FALSE;
   Gen_Protect.stat_Limit_f4 := FALSE;
   Gen_Protect.stat_Limit_f5 := FALSE;
   Gen_Protect.stat_Limit_f6 := FALSE;
   Gen_Protect.stat_Limit_f7 := FALSE;
   Gen_Protect.stat_Limit_f8 := FALSE;
   Gen_Protect.stat_Limit_U1 := FALSE;
   Gen_Protect.stat_Limit_U2 := FALSE;
   Gen_Protect.stat_Limit_U3 := FALSE;
   Gen_Protect.stat_Limit_U4 := FALSE;
   Gen_Protect.stat_Limit_P7_undel := FALSE;
   Gen_Protect.stat_Limit_P7_Warn := FALSE;
   Gen_Protect.stat_ShortCircuit := FALSE;
   Gen_Protect.stat_Wind_Overtemp := FALSE;
   Gen_Protect.stat_Standby_ProtWarn := FALSE;
   Gen_Protect.stat_Uness1_TransfLBrk := FALSE;
   Gen_Protect.stat_ShC_OtherSet_Aux := FALSE;
   Gen_Protect.stat_ShC_OtherSet_Pulse := FALSE;
   Gen_Protect.stat_ShC_OtherSet1 := FALSE;
   Gen_Protect.stat_ShC_OtherSet2 := FALSE;
   Gen_Protect.stat_ShC_OtherSet_Reset := FALSE;
   Gen_Protect.stat_Block_ShC_OtherSet := FALSE;
   Gen_Protect.stat_DiffProt_Trip := FALSE;
   Gen_Protect.stat_Trip_Overcurrent := FALSE;
   Gen_Protect.stat_Trip_RevPower := FALSE;
   Gen_Protect.stat_Trip_Underfrequ := FALSE;
   Gen_Protect.stat_Trip_Undervoltage := FALSE;
   Gen_Protect.stat_Uness2_Uness1 := FALSE;
   Gen_Protect.stat_Uness3_Uness2 := FALSE;
   Gen_Protect.stat_GenRunning := FALSE;
   Gen_Protect.stat_Harb_Feedb_Mode := FALSE;
   Gen_Protect.stat_GENOP_StandbySt := FALSE;
   Gen_Protect.stat_FC56_Limit_01 := FALSE;
   Gen_Protect.stat_FC56_Limit_02 := FALSE;
   Gen_Protect.stat_FC56_Limit_03 := FALSE;
   Gen_Protect.stat_FC56_Limit_04 := FALSE;
   Gen_Protect.stat_FC56_Limit_05 := FALSE;
   Gen_Protect.stat_FC56_Limit_06 := FALSE;
   Gen_Protect.stat_FC56_Limit_07 := FALSE;
   Gen_Protect.stat_FC56_Limit_08 := FALSE;
   Gen_Protect.stat_FC56_Limit_09 := FALSE;
   Gen_Protect.stat_FC56_Limit_10 := FALSE;
   Gen_Protect.stat_FC56_Limit_11 := FALSE;
   Gen_Protect.stat_FC56_Limit_12 := FALSE;
   Gen_Protect.stat_FC56_Limit_13 := FALSE;
   Gen_Protect.stat_FC56_Limit_131 := FALSE;
   Gen_Protect.stat_FC56_Limit_14 := FALSE;
   Gen_Protect.stat_FC56_Limit_15 := FALSE;
   Gen_Protect.stat_FC56_Limit_16 := FALSE;
   Gen_Protect.stat_FC56_Limit_17 := FALSE;
   Gen_Protect.stat_FC56_Limit_18 := FALSE;
   Gen_Protect.stat_FC56_Limit_19 := FALSE;
   Gen_Protect.stat_FC56_Limit_20 := FALSE;
   Gen_Protect.stat_FC56_Limit_21 := FALSE;
   Gen_Protect.stat_FC56_Limit_22 := FALSE;
   Gen_Protect.stat_FC56_Limit_23 := FALSE;
   Gen_Protect.stat_FC56_Limit_24 := FALSE;
   Gen_Protect.stat_FC56_Limit_25 := FALSE;
   Gen_Protect.stat_Underload := FALSE;
   Gen_Protect.stat_UndelayStop := FALSE;
   Gen_Protect.stat_Trip_Temp_Overcurr := FALSE;
   Gen_Breaker.in_DGLoad_off := FALSE;
   Gen_Breaker.in_Nmb_Gen_LoadSh := 0;
   Gen_Breaker.in_act_mode := B#16#0;
   Gen_Breaker.in_EG_Set := FALSE;
   Gen_Breaker.in_Blackout := FALSE;
   Gen_Breaker.in_SimLock_Blocked := FALSE;
   Gen_Breaker.in_SimLock_Fault := FALSE;
   Gen_Breaker.in_SimLock_Release := FALSE;
   Gen_Breaker.in_DGWG_run := FALSE;
   Gen_Breaker.in_DGWG_Stop := FALSE;
   Gen_Breaker.in_GenBrkOff_LoadRed := FALSE;
   Gen_Breaker.in_DGWG_GenBrk_Cmd_Off := FALSE;
   Gen_Breaker.in_DGWG_GenBrk_Cmd_Trip := FALSE;
   Gen_Breaker.in_ChOver_Blackout := FALSE;
   Gen_Breaker.in_Standby_ReadyConn := FALSE;
   Gen_Breaker.in_ShoreConn_Off := FALSE;
   Gen_Breaker.in_DI_GenBrk_ReadyClose := FALSE;
   Gen_Breaker.in_DI_GenBrk_Tripped := FALSE;
   Gen_Breaker.in_DI_GenBrk_PosNorm := FALSE;
   Gen_Breaker.in_DI_GenBrk_PosTest := FALSE;
   Gen_Breaker.in_DI_GenBrk_FB_On := FALSE;
   Gen_Breaker.in_DI_GenBrk_FB_Off := FALSE;
   Gen_Breaker.in_GENOP_SynCmd_On := FALSE;
   Gen_Breaker.in_GenBrk_Ext_Release := FALSE;
   Gen_Breaker.in_ext_DG_block := FALSE;
   Gen_Breaker.in_EG_GB_Close := FALSE;
   Gen_Breaker.in_EG_Cmd_Synchr_On := FALSE;
   Gen_Breaker.in_EG_GB_Open := FALSE;
   Gen_Breaker.in_PB_GenBrk_Close := FALSE;
   Gen_Breaker.in_PB_GenBrk_Open := FALSE;
   Gen_Breaker.in_PB_GenBrk_Open_Man := FALSE;
   Gen_Breaker.in_reset_synchron := FALSE;
   Gen_Breaker.in_Reset := FALSE;
   Gen_Breaker.in_power_avail := FALSE;
   Gen_Breaker.out_Operat_Status := 0;
   Gen_Breaker.out_StandbyStart := FALSE;
   Gen_Breaker.out_SimLock_Request := FALSE;
   Gen_Breaker.out_DO_GenBrk_Cmd_Off := FALSE;
   Gen_Breaker.out_GENOP_GenBrk_Cmd_On := FALSE;
   Gen_Breaker.out_GENOP_GenBrk_Cmd_Off := FALSE;
   Gen_Breaker.out_GENOP_SynchRelease := FALSE;
   Gen_Breaker.out_GenBrk_Ready := FALSE;
   Gen_Breaker.out_GenBrk_Ready_Standby := FALSE;
   Gen_Breaker.out_GenBrk_Ready_Close := FALSE;
   Gen_Breaker.out_Brk_Closed_Plausib := FALSE;
   Gen_Breaker.out_UndelayStop := FALSE;
   Gen_Breaker.out_DelayStop := FALSE;
   Gen_Breaker.out_LoadReduction := FALSE;
   Gen_Breaker.out_Blocking := FALSE;
   Gen_Breaker.out_ChOver_Semi := FALSE;
   Gen_Breaker.out_Fail_Ready := FALSE;
   Gen_Breaker.out_Fail_FeedbOn := FALSE;
   Gen_Breaker.out_Fail_FeedbOff := FALSE;
   Gen_Breaker.out_Fail_FeedbOffOn := FALSE;
   Gen_Breaker.out_Fail_BrkTrip := FALSE;
   Gen_Breaker.out_Fail_SynTime := FALSE;
   Gen_Breaker.out_Fail_GenFailure := FALSE;
   Gen_Breaker.out_Fail_ShoreC_GenBrk := FALSE;
   Gen_Breaker.out_Fail_ChgViaBlack := FALSE;
   Gen_Breaker.stat_CntValue01 := 0;
   Gen_Breaker.stat_CntValue02 := 0;
   Gen_Breaker.stat_CntValue03 := 0;
   Gen_Breaker.stat_CntValue04 := 0;
   Gen_Breaker.stat_CntValue05 := 0;
   Gen_Breaker.stat_CntValue06 := 0;
   Gen_Breaker.stat_CntValue07 := 0;
   Gen_Breaker.stat_CntValue08 := 0;
   Gen_Breaker.stat_CntValue09 := 0;
   Gen_Breaker.stat_CntValue10 := 0;
   Gen_Breaker.stat_CntValue11 := 0;
   Gen_Breaker.stat_CntValue12 := 0;
   Gen_Breaker.stat_CntValue13 := 0;
   Gen_Breaker.stat_CntValue14 := 0;
   Gen_Breaker.stat_CntStart01 := FALSE;
   Gen_Breaker.stat_CntStarted01 := FALSE;
   Gen_Breaker.stat_CntStart02 := FALSE;
   Gen_Breaker.stat_CntStarted02 := FALSE;
   Gen_Breaker.stat_CntStart03 := FALSE;
   Gen_Breaker.stat_CntStarted03 := FALSE;
   Gen_Breaker.stat_CntStart04 := FALSE;
   Gen_Breaker.stat_CntStarted04 := FALSE;
   Gen_Breaker.stat_CntStart05 := FALSE;
   Gen_Breaker.stat_CntStarted05 := FALSE;
   Gen_Breaker.stat_CntStart06 := FALSE;
   Gen_Breaker.stat_CntStarted06 := FALSE;
   Gen_Breaker.stat_CntStart07 := FALSE;
   Gen_Breaker.stat_CntStarted07 := FALSE;
   Gen_Breaker.stat_CntStart08 := FALSE;
   Gen_Breaker.stat_CntStarted08 := FALSE;
   Gen_Breaker.stat_CntStart09 := FALSE;
   Gen_Breaker.stat_CntStarted09 := FALSE;
   Gen_Breaker.stat_CntStart10 := FALSE;
   Gen_Breaker.stat_CntStarted10 := FALSE;
   Gen_Breaker.stat_CntStart11 := FALSE;
   Gen_Breaker.stat_CntStarted11 := FALSE;
   Gen_Breaker.stat_CntStart12 := FALSE;
   Gen_Breaker.stat_CntStarted12 := FALSE;
   Gen_Breaker.stat_CntStart13 := FALSE;
   Gen_Breaker.stat_CntStarted13 := FALSE;
   Gen_Breaker.stat_CntStart14 := FALSE;
   Gen_Breaker.stat_CntStarted14 := FALSE;
   Gen_Breaker.stat_BrkReady_TimeEx := FALSE;
   Gen_Breaker.stat_BrkClose_Semi := FALSE;
   Gen_Breaker.stat_BrkOn_Sim := FALSE;
   Gen_Breaker.stat_SynchOn_Pulse := FALSE;
   Gen_Breaker.stat_SynchOn_EG_PAux := FALSE;
   Gen_Breaker.stat_SynchOn := FALSE;
   Gen_Breaker.stat_Synch_TimeEx := FALSE;
   Gen_Breaker.stat_GenBrk_Off_NoLoadR := FALSE;
   Gen_Breaker.stat_GenBrk_Off_LoadRed := FALSE;
   Gen_Breaker.stat_LoadRed_TimeEx := FALSE;
   Gen_Breaker.stat_GenBrkOff_Limit := FALSE;
   Gen_Breaker.stat_GenBrkOff_StbyReady := FALSE;
   Gen_Breaker.stat_FeedbOn_TimeSt := FALSE;
   Gen_Breaker.stat_FeedbOn_TimeEx := FALSE;
   Gen_Breaker.stat_FeedbOff_TimeSt := FALSE;
   Gen_Breaker.stat_FeedbOff_TimeEx := FALSE;
   Gen_Breaker.stat_GenBrk_DelayOff := FALSE;
   Gen_Breaker.stat_PulseAux_Trip := FALSE;
   Gen_Breaker.stat_Fail_GenBrk := FALSE;
   Gen_Breaker.stat_Fail_ShoreC := FALSE;
   Gen_Breaker.stat_synchron := FALSE;
   Gen_Breaker.stat_Fail_GenBrk_TripExt := FALSE;
   Gen_Breaker.stat_PulseAux_GenBrk_Off := FALSE;
   Gen_Breaker.stat_Fail_GenBrk_TripNoR := FALSE;
   Gen_Breaker.stat_GENOP_GenBrk_CmdOff := FALSE;
   Gen_Breaker.stat_power_avail := FALSE;
   RemoteStart.IN_start := FALSE;
   RemoteStart.IN_destGen := B#16#0;
   RemoteStart.IN_time := S5T#0MS;
   RemoteStart.IN_timerNo := T 0;
   RemoteStart.OUT_sendPulse := FALSE;
   RemoteStart.stat_step := B#16#0;
   RemoteStart.stat_destGen := B#16#0;
   RemoteStart.stat_startPulse := FALSE;
   RemoteStart.stat_sendSignal := FALSE;
   RemoteStart.stat_pulseStep1 := FALSE;
   RemoteStart.stat_pulseStep2 := FALSE;
   BlockTieBrk := FALSE;
   BothSideBlackout := FALSE;
   tieBrk_state := FALSE;
   pulse_SlvBrk := FALSE;
   Generator_Protect.in_GEN_I_L1 := 0;
   Generator_Protect.in_GEN_I_L2 := 0;
   Generator_Protect.in_GEN_I_L3 := 0;
   Generator_Protect.in_GEN_P_SUM := 0;
   Generator_Protect.in_BUS_f := 0;
   Generator_Protect.in_BUS_U_L1L2 := 0;
   Generator_Protect.in_BUS_U_L2L3 := 0;
   Generator_Protect.in_BUS_U_L3L1 := 0;
   Generator_Protect.in_GEN_U_L1L2 := 0;
   Generator_Protect.in_GEN_U_L2L3 := 0;
   Generator_Protect.in_GEN_U_L3L1 := 0;
   Generator_Protect.in_Nmb_Generator := 0;
   Generator_Protect.in_act_mode := B#16#0;
   Generator_Protect.in_EG_Set := FALSE;
   Generator_Protect.in_EG_Harbour_Mode := FALSE;
   Generator_Protect.in_EG_PowerFb_Mode := FALSE;
   Generator_Protect.in_DI_Blackout := FALSE;
   Generator_Protect.in_DI_BusbarVolt := FALSE;
   Generator_Protect.in_DI_FireSpeedRelGenBrk := FALSE;
   Generator_Protect.in_DI_FB_GenBrk_On := FALSE;
   Generator_Protect.in_DI_Wind_Overtemp := FALSE;
   Generator_Protect.in_DiffProt_warn := FALSE;
   Generator_Protect.in_DiffProt_Trip := FALSE;
   Generator_Protect.in_Overc_ShortC_extern := FALSE;
   Generator_Protect.in_GENOP_ShortCircuit := FALSE;
   Generator_Protect.in_GENOP_Overcurrent := FALSE;
   Generator_Protect.in_GENOP_ReversePower := FALSE;
   Generator_Protect.in_GENOP_Unessent1 := FALSE;
   Generator_Protect.in_GENOP_Unessent2 := FALSE;
   Generator_Protect.in_GENOP_Unessent3 := FALSE;
   Generator_Protect.in_Rel_UnderlShd := FALSE;
   Generator_Protect.in_UnderShd_pos := FALSE;
   Generator_Protect.in_ShortCirc_OtherGen := FALSE;
   Generator_Protect.in_Reset := FALSE;
   Generator_Protect.in_p_uncond_reset := FALSE;
   Generator_Protect.out_Blackout := FALSE;
   Generator_Protect.out_BusVolt_avail := FALSE;
   Generator_Protect.out_GenVolt_avail := FALSE;
   Generator_Protect.out_StandbyStart := FALSE;
   Generator_Protect.out_Uness1_Off := FALSE;
   Generator_Protect.out_Uness2_Off := FALSE;
   Generator_Protect.out_Uness3_Off := FALSE;
   Generator_Protect.out_GenBrk_Off := FALSE;
   Generator_Protect.out_ShortCirc_OtherGen := FALSE;
   Generator_Protect.out_VoltContr_Off := FALSE;
   Generator_Protect.out_UndelayStop := FALSE;
   Generator_Protect.out_Blocking := FALSE;
   Generator_Protect.out_ChOver_Semi := FALSE;
   Generator_Protect.out_ChOver_Blackout := FALSE;
   Generator_Protect.out_Underload_Limit := FALSE;
   Generator_Protect.out_Underload_Shd := FALSE;
   Generator_Protect.out_Fail_Busbar := FALSE;
   Generator_Protect.out_Fail_Current := FALSE;
   Generator_Protect.out_Fail_Overcurr := FALSE;
   Generator_Protect.out_Fail_shortCirc := FALSE;
   Generator_Protect.out_Fail_RevPower := FALSE;
   Generator_Protect.out_Fail_overcurrent := FALSE;
   Generator_Protect.out_Fail_overload := FALSE;
   Generator_Protect.out_Fail_Underfrequ1 := FALSE;
   Generator_Protect.out_Fail_Underfrequ2 := FALSE;
   Generator_Protect.out_Fail_Underfrequ3 := FALSE;
   Generator_Protect.out_Fail_Overfrequ := FALSE;
   Generator_Protect.out_Fail_Undervolt1 := FALSE;
   Generator_Protect.out_Fail_Undervolt2 := FALSE;
   Generator_Protect.out_Fail_Overvolt1 := FALSE;
   Generator_Protect.out_Fail_Overvolt2 := FALSE;
   Generator_Protect.out_Fail_ShortCirc_Other := FALSE;
   Generator_Protect.out_Fail_DiffProt_Warn := FALSE;
   Generator_Protect.out_Fail_DiffProt_Trip := FALSE;
   Generator_Protect.out_Fail_Wind_Overtemp := FALSE;
   Generator_Protect.out_Fail_Underload := FALSE;
   Generator_Protect.out_Fail_Underl_SD := FALSE;
   Generator_Protect.out_Spare_1 := FALSE;
   Generator_Protect.out_Spare_2 := FALSE;
   Generator_Protect.out_PrtcEG_sign := DW#16#0;
   Generator_Protect.stat_GEN_I_Min := 0;
   Generator_Protect.stat_GEN_I_Max := 0;
   Generator_Protect.stat_GEN_I_Mean := 0;
   Generator_Protect.stat_BUS_U_Min := 0;
   Generator_Protect.stat_BUS_U_Max := 0;
   Generator_Protect.stat_GEN_U_Min := 0;
   Generator_Protect.stat_GEN_U_Max := 0;
   Generator_Protect.stat_Limit_I1 := FALSE;
   Generator_Protect.stat_Limit_I2 := FALSE;
   Generator_Protect.stat_Limit_I3 := FALSE;
   Generator_Protect.stat_Limit_I4 := FALSE;
   Generator_Protect.stat_Limit_I5 := FALSE;
   Generator_Protect.stat_Limit_I6 := FALSE;
   Generator_Protect.stat_Limit_I7 := FALSE;
   Generator_Protect.stat_Limit_P1 := FALSE;
   Generator_Protect.stat_Limit_P2 := FALSE;
   Generator_Protect.stat_Limit_P3 := FALSE;
   Generator_Protect.stat_Limit_P4 := FALSE;
   Generator_Protect.stat_Limit_P5 := FALSE;
   Generator_Protect.stat_Limit_P6 := FALSE;
   Generator_Protect.stat_Limit_P7 := FALSE;
   Generator_Protect.stat_Limit_f1 := FALSE;
   Generator_Protect.stat_Limit_f2 := FALSE;
   Generator_Protect.stat_Limit_f3 := FALSE;
   Generator_Protect.stat_Limit_f4 := FALSE;
   Generator_Protect.stat_Limit_f5 := FALSE;
   Generator_Protect.stat_Limit_f6 := FALSE;
   Generator_Protect.stat_Limit_f7 := FALSE;
   Generator_Protect.stat_Limit_f8 := FALSE;
   Generator_Protect.stat_Limit_U1 := FALSE;
   Generator_Protect.stat_Limit_U2 := FALSE;
   Generator_Protect.stat_Limit_U3 := FALSE;
   Generator_Protect.stat_Limit_U4 := FALSE;
   Generator_Protect.stat_Limit_P7_undel := FALSE;
   Generator_Protect.stat_Limit_P7_Warn := FALSE;
   Generator_Protect.stat_ShortCircuit := FALSE;
   Generator_Protect.stat_Wind_Overtemp := FALSE;
   Generator_Protect.stat_Standby_ProtWarn := FALSE;
   Generator_Protect.stat_Uness1_TransfLBrk := FALSE;
   Generator_Protect.stat_ShC_OtherSet_Aux := FALSE;
   Generator_Protect.stat_ShC_OtherSet_Pulse := FALSE;
   Generator_Protect.stat_ShC_OtherSet1 := FALSE;
   Generator_Protect.stat_ShC_OtherSet2 := FALSE;
   Generator_Protect.stat_ShC_OtherSet_Reset := FALSE;
   Generator_Protect.stat_Block_ShC_OtherSet := FALSE;
   Generator_Protect.stat_DiffProt_Trip := FALSE;
   Generator_Protect.stat_Trip_Overcurrent := FALSE;
   Generator_Protect.stat_Trip_RevPower := FALSE;
   Generator_Protect.stat_Trip_Underfrequ := FALSE;
   Generator_Protect.stat_Trip_Undervoltage := FALSE;
   Generator_Protect.stat_Uness2_Uness1 := FALSE;
   Generator_Protect.stat_Uness3_Uness2 := FALSE;
   Generator_Protect.stat_GenRunning := FALSE;
   Generator_Protect.stat_Harb_Feedb_Mode := FALSE;
   Generator_Protect.stat_GENOP_StandbySt := FALSE;
   Generator_Protect.stat_FC56_Limit_01 := FALSE;
   Generator_Protect.stat_FC56_Limit_02 := FALSE;
   Generator_Protect.stat_FC56_Limit_03 := FALSE;
   Generator_Protect.stat_FC56_Limit_04 := FALSE;
   Generator_Protect.stat_FC56_Limit_05 := FALSE;
   Generator_Protect.stat_FC56_Limit_06 := FALSE;
   Generator_Protect.stat_FC56_Limit_07 := FALSE;
   Generator_Protect.stat_FC56_Limit_08 := FALSE;
   Generator_Protect.stat_FC56_Limit_09 := FALSE;
   Generator_Protect.stat_FC56_Limit_10 := FALSE;
   Generator_Protect.stat_FC56_Limit_11 := FALSE;
   Generator_Protect.stat_FC56_Limit_12 := FALSE;
   Generator_Protect.stat_FC56_Limit_13 := FALSE;
   Generator_Protect.stat_FC56_Limit_131 := FALSE;
   Generator_Protect.stat_FC56_Limit_14 := FALSE;
   Generator_Protect.stat_FC56_Limit_15 := FALSE;
   Generator_Protect.stat_FC56_Limit_16 := FALSE;
   Generator_Protect.stat_FC56_Limit_17 := FALSE;
   Generator_Protect.stat_FC56_Limit_18 := FALSE;
   Generator_Protect.stat_FC56_Limit_19 := FALSE;
   Generator_Protect.stat_FC56_Limit_20 := FALSE;
   Generator_Protect.stat_FC56_Limit_21 := FALSE;
   Generator_Protect.stat_FC56_Limit_22 := FALSE;
   Generator_Protect.stat_FC56_Limit_23 := FALSE;
   Generator_Protect.stat_FC56_Limit_24 := FALSE;
   Generator_Protect.stat_FC56_Limit_25 := FALSE;
   Generator_Protect.stat_Underload := FALSE;
   Generator_Protect.stat_UndelayStop := FALSE;
   Generator_Protect.stat_Trip_Temp_Overcurr := FALSE;
   Breaker_control.in_DGLoad_off := FALSE;
   Breaker_control.in_Nmb_Gen_LoadSh := 0;
   Breaker_control.in_act_mode := B#16#0;
   Breaker_control.in_EG_Set := FALSE;
   Breaker_control.in_Blackout := FALSE;
   Breaker_control.in_SimLock_Blocked := FALSE;
   Breaker_control.in_SimLock_Fault := FALSE;
   Breaker_control.in_SimLock_Release := FALSE;
   Breaker_control.in_DGWG_run := FALSE;
   Breaker_control.in_DGWG_Stop := FALSE;
   Breaker_control.in_GenBrkOff_LoadRed := FALSE;
   Breaker_control.in_DGWG_GenBrk_Cmd_Off := FALSE;
   Breaker_control.in_DGWG_GenBrk_Cmd_Trip := FALSE;
   Breaker_control.in_ChOver_Blackout := FALSE;
   Breaker_control.in_Standby_ReadyConn := FALSE;
   Breaker_control.in_ShoreConn_Off := FALSE;
   Breaker_control.in_DI_GenBrk_ReadyClose := FALSE;
   Breaker_control.in_DI_GenBrk_Tripped := FALSE;
   Breaker_control.in_DI_GenBrk_PosNorm := FALSE;
   Breaker_control.in_DI_GenBrk_PosTest := FALSE;
   Breaker_control.in_DI_GenBrk_FB_On := FALSE;
   Breaker_control.in_DI_GenBrk_FB_Off := FALSE;
   Breaker_control.in_GENOP_SynCmd_On := FALSE;
   Breaker_control.in_GenBrk_Ext_Release := FALSE;
   Breaker_control.in_ext_DG_block := FALSE;
   Breaker_control.in_EG_GB_Close := FALSE;
   Breaker_control.in_EG_Cmd_Synchr_On := FALSE;
   Breaker_control.in_EG_GB_Open := FALSE;
   Breaker_control.in_PB_GenBrk_Close := FALSE;
   Breaker_control.in_PB_GenBrk_Open := FALSE;
   Breaker_control.in_PB_GenBrk_Open_Man := FALSE;
   Breaker_control.in_reset_synchron := FALSE;
   Breaker_control.in_Reset := FALSE;
   Breaker_control.in_power_avail := FALSE;
   Breaker_control.out_Operat_Status := 0;
   Breaker_control.out_StandbyStart := FALSE;
   Breaker_control.out_SimLock_Request := FALSE;
   Breaker_control.out_DO_GenBrk_Cmd_Off := FALSE;
   Breaker_control.out_GENOP_GenBrk_Cmd_On := FALSE;
   Breaker_control.out_GENOP_GenBrk_Cmd_Off := FALSE;
   Breaker_control.out_GENOP_SynchRelease := FALSE;
   Breaker_control.out_GenBrk_Ready := FALSE;
   Breaker_control.out_GenBrk_Ready_Standby := FALSE;
   Breaker_control.out_GenBrk_Ready_Close := FALSE;
   Breaker_control.out_Brk_Closed_Plausib := FALSE;
   Breaker_control.out_UndelayStop := FALSE;
   Breaker_control.out_DelayStop := FALSE;
   Breaker_control.out_LoadReduction := FALSE;
   Breaker_control.out_Blocking := FALSE;
   Breaker_control.out_ChOver_Semi := FALSE;
   Breaker_control.out_Fail_Ready := FALSE;
   Breaker_control.out_Fail_FeedbOn := FALSE;
   Breaker_control.out_Fail_FeedbOff := FALSE;
   Breaker_control.out_Fail_FeedbOffOn := FALSE;
   Breaker_control.out_Fail_BrkTrip := FALSE;
   Breaker_control.out_Fail_SynTime := FALSE;
   Breaker_control.out_Fail_GenFailure := FALSE;
   Breaker_control.out_Fail_ShoreC_GenBrk := FALSE;
   Breaker_control.out_Fail_ChgViaBlack := FALSE;
   Breaker_control.stat_CntValue01 := 0;
   Breaker_control.stat_CntValue02 := 0;
   Breaker_control.stat_CntValue03 := 0;
   Breaker_control.stat_CntValue04 := 0;
   Breaker_control.stat_CntValue05 := 0;
   Breaker_control.stat_CntValue06 := 0;
   Breaker_control.stat_CntValue07 := 0;
   Breaker_control.stat_CntValue08 := 0;
   Breaker_control.stat_CntValue09 := 0;
   Breaker_control.stat_CntValue10 := 0;
   Breaker_control.stat_CntValue11 := 0;
   Breaker_control.stat_CntValue12 := 0;
   Breaker_control.stat_CntValue13 := 0;
   Breaker_control.stat_CntValue14 := 0;
   Breaker_control.stat_CntStart01 := FALSE;
   Breaker_control.stat_CntStarted01 := FALSE;
   Breaker_control.stat_CntStart02 := FALSE;
   Breaker_control.stat_CntStarted02 := FALSE;
   Breaker_control.stat_CntStart03 := FALSE;
   Breaker_control.stat_CntStarted03 := FALSE;
   Breaker_control.stat_CntStart04 := FALSE;
   Breaker_control.stat_CntStarted04 := FALSE;
   Breaker_control.stat_CntStart05 := FALSE;
   Breaker_control.stat_CntStarted05 := FALSE;
   Breaker_control.stat_CntStart06 := FALSE;
   Breaker_control.stat_CntStarted06 := FALSE;
   Breaker_control.stat_CntStart07 := FALSE;
   Breaker_control.stat_CntStarted07 := FALSE;
   Breaker_control.stat_CntStart08 := FALSE;
   Breaker_control.stat_CntStarted08 := FALSE;
   Breaker_control.stat_CntStart09 := FALSE;
   Breaker_control.stat_CntStarted09 := FALSE;
   Breaker_control.stat_CntStart10 := FALSE;
   Breaker_control.stat_CntStarted10 := FALSE;
   Breaker_control.stat_CntStart11 := FALSE;
   Breaker_control.stat_CntStarted11 := FALSE;
   Breaker_control.stat_CntStart12 := FALSE;
   Breaker_control.stat_CntStarted12 := FALSE;
   Breaker_control.stat_CntStart13 := FALSE;
   Breaker_control.stat_CntStarted13 := FALSE;
   Breaker_control.stat_CntStart14 := FALSE;
   Breaker_control.stat_CntStarted14 := FALSE;
   Breaker_control.stat_BrkReady_TimeEx := FALSE;
   Breaker_control.stat_BrkClose_Semi := FALSE;
   Breaker_control.stat_BrkOn_Sim := FALSE;
   Breaker_control.stat_SynchOn_Pulse := FALSE;
   Breaker_control.stat_SynchOn_EG_PAux := FALSE;
   Breaker_control.stat_SynchOn := FALSE;
   Breaker_control.stat_Synch_TimeEx := FALSE;
   Breaker_control.stat_GenBrk_Off_NoLoadR := FALSE;
   Breaker_control.stat_GenBrk_Off_LoadRed := FALSE;
   Breaker_control.stat_LoadRed_TimeEx := FALSE;
   Breaker_control.stat_GenBrkOff_Limit := FALSE;
   Breaker_control.stat_GenBrkOff_StbyReady := FALSE;
   Breaker_control.stat_FeedbOn_TimeSt := FALSE;
   Breaker_control.stat_FeedbOn_TimeEx := FALSE;
   Breaker_control.stat_FeedbOff_TimeSt := FALSE;
   Breaker_control.stat_FeedbOff_TimeEx := FALSE;
   Breaker_control.stat_GenBrk_DelayOff := FALSE;
   Breaker_control.stat_PulseAux_Trip := FALSE;
   Breaker_control.stat_Fail_GenBrk := FALSE;
   Breaker_control.stat_Fail_ShoreC := FALSE;
   Breaker_control.stat_synchron := FALSE;
   Breaker_control.stat_Fail_GenBrk_TripExt := FALSE;
   Breaker_control.stat_PulseAux_GenBrk_Off := FALSE;
   Breaker_control.stat_Fail_GenBrk_TripNoR := FALSE;
   Breaker_control.stat_GENOP_GenBrk_CmdOff := FALSE;
   Breaker_control.stat_power_avail := FALSE;
   memo_GenSetOnBus := W#16#0;
   memo_newGenSet := W#16#0;
END_DATA_BLOCK



FUNCTION "fc_TieBrk_one" : VOID
TITLE =Control of one tie breaker
//version!date    !author !change_segm!change_description
//-------+--------+-------+-----------+-------------------------------
// 1.0   !04.10.00!Kahle  ! ---       ! 1st valid version
// 1.1   !13.10.00!Kahle  ! 2         ! new parameter 'IN_othBrk_on'
// 1.2   !20.10.00!Kahle  ! 2         ! close brk aft.blackout if no EG mode only
//       !        !       ! 5         ! corr.parameter 'FDB_close_B'
// 1.3   !14.11.00!Kahle  ! 2         ! add.signal "slave breaker"
//       !        !       !           ! in case of blackout open breaker
//       !        !       !           ! ext.blocking ->norm position
// 1.4   !11.01.01!Kahle  ! 5         ! Corr. breaker on in case of blackout
//       !        !       ! 6,7(new)  ! blocking tie breaker off
// 1.5   !14.03.01!Kahle  ! 2         ! New alarms "overcurrent","overload"
AUTHOR : Kahle
FAMILY : PMA71
NAME : Tie2Ctrl
VERSION : 1.5


VAR_TEMP
  c_lockCtrl_1 : BOOL ;	//command: lock controller (from program I)
  c_simLock_1 : BOOL ;	//command: simultanoeus lock (from program I)
  c_reqStart : BOOL ;	//command: request next generator set (from program I)
  f_I_sc_1 : BOOL ;	//feedback: short circuit detected (from program I)
  c_lockCtrl_2 : BOOL ;	//command: lock controller (from program II)
  c_simLock_2 : BOOL ;	//command: simultanoeus lock (from program II)
  c_reqStart2 : BOOL ;	//command: request next generator set (from program II)
  f_I_sc_2 : BOOL ;	//feedback: short circuit detected (from program II)
  stdbyNo_1 : BYTE ;	//Number of the actual standby set (from program I)
  stdbyNo_2 : BYTE ;	//Number of the actual standby set (from program II)
  synchr_1 : BOOL ;	//Synchronizing active (tie breaker A)
  synchr_2 : BOOL ;	//Synchronizing active (tie breaker B)
  block_1 : BOOL ;	//Tie breaker 1 is blocked
  block_2 : BOOL ;	//Tie breaker 2 is blocked
  shortCirc_1 : BOOL ;	//Tie breaker 1 short circuit dedected
  shortCirc_2 : BOOL ;	//Tie breaker 2 short circuit dedected
  shoreConn_1 : BOOL ;	//shore connection A is active
  shoreConn_2 : BOOL ;	//shore connection B is active
  Blackout_busbar : BOOL ;	//Blackout busbar
  Blackout_trans : BOOL ;	//Blackout transferline
  BothShoreExp : BOOL ;	//Both shore connection are in export direction
  cfgBusbar : INT ;	//Actual configuration busbar
  total_CfgBusbar : DWORD ;	//Total actual configuration busbar
  f_auto_tb : BOOL ;	//received feedback configuration busbar
  f_rdyStdby_tb : BOOL ;	//received feedback configuration busbar
  f_brk_clse_tb : BOOL ;	//received feedback configuration busbar
  f_onbus_tb : BOOL ;	//received feedback configuration busbar
  f_lock_tb : BOOL ;	//received feedback configuration busbar
  f_run_tb : BOOL ;	//received feedback configuration busbar
  f_blackout_tb : BOOL ;	//received feedback configuration busbar
  f_SGonbus_tb : BOOL ;	//received feedback configuration busbar
END_VAR
BEGIN
NETWORK
TITLE =Shore connection blocked if direction =export
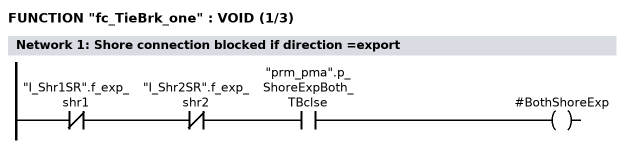
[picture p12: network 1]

      UN    "I_Shr1SR".f_exp_shr1;
      UN    "I_Shr2SR".f_exp_shr2;
      U     "prm_pma".p_ShoreExpBoth_TBclse;
      =     #BothShoreExp;
NETWORK
TITLE =Control tie breaker No.1
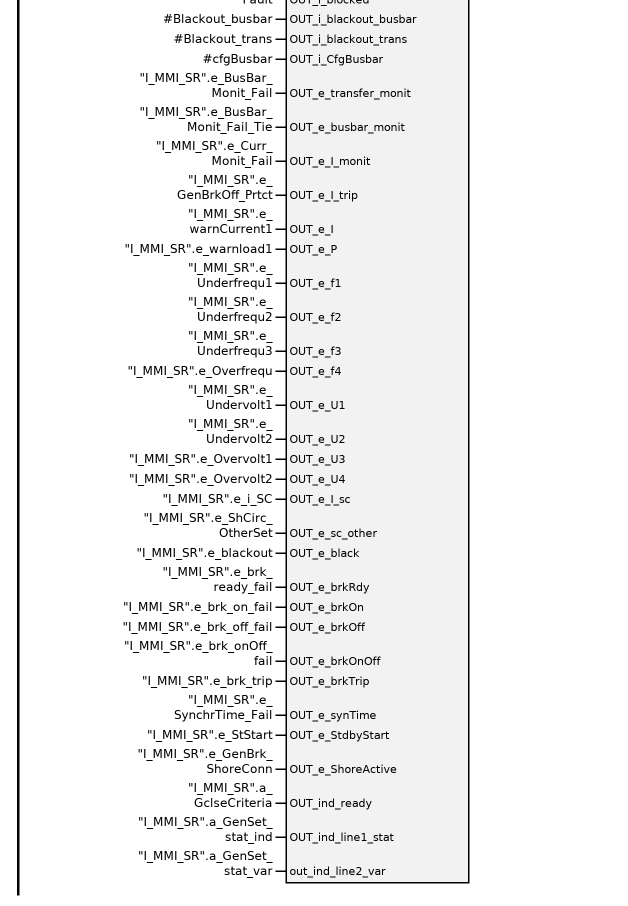
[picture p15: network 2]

      U     "prm_pma".p_invAllocation;
      =     L     13.0;
      BLD   103;
      U(    ;
      O     "I_MMI_SR".c_genBrk_clse;
      O     ;
      U     "MEM".o520_closeBrk_A;
      U(    ;
      ON    "MEM".o515R_f_EB_busbar;
      ON    "prm_pma".p_TrsLine;
      )     ;
      )     ;
      =     L     13.1;
      BLD   103;
      U(    ;
      U     "I_MMI_SR".c_genBrk_opn;
      UN    "MEM".o520_blockTBopn;
      O(    ;
      U(    ;
      U     "IN_black_trs";
      UN    "IN_non_black_trs";
      O     ;
      U     "IN_black_bus";
      UN    "IN_non_black_bus";
      )     ;
      FP    "p_SlvBrk_off";
      U     "prm_pma".p_TieBrkOnBlack;
      )     ;
      )     ;
      =     L     13.2;
      BLD   103;
      U     "IN_PB_TieBrk_Off";
      =     L     13.3;
      BLD   103;
      U     "IN_black_bus";
      =     L     13.4;
      BLD   103;
      U     "IN_non_black_bus";
      =     L     13.5;
      BLD   103;
      U     "IN_black_trs";
      =     L     13.6;
      BLD   103;
      U     "IN_non_black_trs";
      =     L     13.7;
      BLD   103;
      U     "IN_SlvBrk_clse";
      UN    "IN_SlvBrk_opn";
      =     L     14.0;
      BLD   103;
      U(    ;
      O     "IN_shore_clse_bus";
      O     "I_Shr1SR".f_brk_clse;
      )     ;
      =     L     14.1;
      BLD   103;
      U(    ;
      O     "IN_shore_clse_trs";
      O     "I_Shr2SR".f_brk_clse;
      )     ;
      =     L     14.2;
      BLD   103;
      U     #BothShoreExp;
      =     L     14.3;
      BLD   103;
      U(    ;
      O     "MEM".o515R_f_i_SC;
      O     "i_shortCirc_2ndBrk";
      )     ;
      =     L     14.4;
      BLD   103;
      U     "IN_brk_Tripped";
      =     L     14.5;
      BLD   103;
      U     "I_prtcSR".e_I_SC_VER;
      =     L     14.6;
      BLD   103;
      U     "I_prtcSR".e_I_GW1VER;
      =     L     14.7;
      BLD   103;
      U     "I_prtcSR".e_I_GW2VER;
      =     L     15.0;
      BLD   103;
      U     "I_prtcSR".e_I_GW3VER;
      =     L     15.1;
      BLD   103;
      U     "I_prtcSR".e_I_GW4VER;
      =     L     15.2;
      BLD   103;
      U     "MEM".o515_ownBlock;
      =     L     15.3;
      BLD   103;
      U     "MEM".o515_simulLockErr;
      =     L     15.4;
      BLD   103;
      U     "MEM".o515_simulLockAct;
      =     L     15.5;
      BLD   103;
      U     "IN_brk_normPos";
      =     L     15.6;
      BLD   103;
      U     "IN_brk_normPos";
      UN    "MEM".o57_extBlock;
      =     L     15.7;
      BLD   103;
      U     "IN_brk_testPos";
      =     L     16.0;
      BLD   103;
      U     "IN_brk_clse";
      =     L     16.1;
      BLD   103;
      U     "IN_brk_opn";
      =     L     16.2;
      BLD   103;
      U     "false";
      =     L     16.3;
      BLD   103;
      U     "I_prtcSR".i_BR_ON;
      =     L     16.4;
      BLD   103;
      U     "I_MMI_SR".c_rst_alm;
      =     L     16.5;
      BLD   103;
      U     "MEM".o51_blockF_reset;
      =     L     16.6;
      BLD   103;
      U     "MEM".o51_i_pressCnfrm;
      =     L     16.7;
      BLD   103;
      U     "true";
      SPBNB _007;
      CALL "fb_520_tieBreaker" , "tieB_1" (
           IN_synchrToOwnBus        := L     13.0,
           IN_cmd_TieBrk_on         := L     13.1,
           IN_cmd_TieBrk_off        := L     13.2,
           IN_PB_TieBrk_off         := L     13.3,
           IN_blackout_bus          := L     13.4,
           IN_VoltAvail_bus         := L     13.5,
           IN_blackout_TRS          := L     13.6,
           IN_VoltAvail_TRS         := L     13.7,
           IN_slaveBrk_on           := L     14.0,
           IN_shoreConnBus_active   := L     14.1,
           IN_shoreConnTrs_active   := L     14.2,
           IN_both_shore_exp        := L     14.3,
           IN_shortCircuit_otherG   := L     14.4,
           IN_shortCircuit_ext      := L     14.5,
           IN_GEN_I_L1              := "I_prtcSR".a_I_L1,
           IN_GEN_I_L2              := "I_prtcSR".a_I_L2,
           IN_GEN_I_L3              := "I_prtcSR".a_I_L3,
           IN_LOAD                  := "I_prtcSR".a_P_SUM,
           IN_BUS_f                 := "I_prtcSR".a_FREQ_BUS,
           IN_GEN_f                 := "I_prtcSR".a_FREQ_GEN,
           IN_BUS_U_L1L2            := "I_prtcSR".a_BUS_L1_L2,
           IN_BUS_U_L2L3            := "I_prtcSR".a_BUS_L2_L3,
           IN_BUS_U_L1L3            := "I_prtcSR".a_BUS_L1_L3,
           IN_GEN_U_L1L21           := "I_prtcSR".a_GEN_L1_L2,
           IN_GEN_U_L2L31           := "I_prtcSR".a_GEN_L2_L3,
           IN_GEN_U_L1L31           := "I_prtcSR".a_GEN_L1_L3,
           IN_I_SC_GW1              := L     14.6,
           IN_I_GW1VER              := L     14.7,
           IN_I_GW2VER              := L     15.0,
           IN_I_GW3VER              := L     15.1,
           IN_I_GW4VER              := L     15.2,
           IN_simLock_blc           := L     15.3,
           IN_simLock_err           := L     15.4,
           IN_simLockRel            := L     15.5,
           IN_brk_ready             := L     15.6,
           IN_brk_normPos           := L     15.7,
           IN_brk_testPos           := L     16.0,
           IN_brk_on                := L     16.1,
           IN_brk_off               := L     16.2,
           IN_othBrk_on             := L     16.3,
           IN_f_cmdBrkOn            := L     16.4,
           IN_reset                 := L     16.5,
           IN_resetBlock            := L     16.6,
           IN_pressCnfrm            := L     16.7,
           IN_mode                  := "MEM".o51_mode_bin,
           IN_TimerStdbyStrt        := "dlyT_StdByStrt_tieBrkA",
           IN_TimerOpnBrk4Gen       := "dlyT_OpnTieBrk_A",
           OUT_SynchrActive         := "OUT_synchrActive",
           OUT_c_LckCtrl            := "MEM".o515_c_LckCtrl,
           OUT_c_simLock            := "MEM".o515_c_simulLock,
           OUT_c_brkON              := "I_prtcSR".c_BR_ON,
           OUT_c_brkOFF             := "I_prtcSR".c_BR_OFF,
           OUT_c_synRel             := "I_prtcSR".c_SYN_EN,
           OUT_c_reqStrt            := "MEM".o515_c_reqStrt,
           OUT_c_sc_otherSet        := "MEM".o515_f_i_SC,
           OUT_i_blocked            := "MEM".o53_Blocked_Fault,
           OUT_i_blackout_busbar    := #Blackout_busbar,
           OUT_i_blackout_trans     := #Blackout_trans,
           OUT_i_CfgBusbar          := #cfgBusbar,
           OUT_e_transfer_monit     := "I_MMI_SR".e_BusBar_Monit_Fail,
           OUT_e_busbar_monit       := "I_MMI_SR".e_BusBar_Monit_Fail_Tie,
           OUT_e_I_monit            := "I_MMI_SR".e_Curr_Monit_Fail,
           OUT_e_I_trip             := "I_MMI_SR".e_GenBrkOff_Prtct,
           OUT_e_I                  := "I_MMI_SR".e_warnCurrent1,
           OUT_e_P                  := "I_MMI_SR".e_warnload1,
           OUT_e_f1                 := "I_MMI_SR".e_Underfrequ1,
           OUT_e_f2                 := "I_MMI_SR".e_Underfrequ2,
           OUT_e_f3                 := "I_MMI_SR".e_Underfrequ3,
           OUT_e_f4                 := "I_MMI_SR".e_Overfrequ,
           OUT_e_U1                 := "I_MMI_SR".e_Undervolt1,
           OUT_e_U2                 := "I_MMI_SR".e_Undervolt2,
           OUT_e_U3                 := "I_MMI_SR".e_Overvolt1,
           OUT_e_U4                 := "I_MMI_SR".e_Overvolt2,
           OUT_e_I_sc               := "I_MMI_SR".e_i_SC,
           OUT_e_sc_other           := "I_MMI_SR".e_ShCirc_OtherSet,
           OUT_e_black              := "I_MMI_SR".e_blackout,
           OUT_e_brkRdy             := "I_MMI_SR".e_brk_ready_fail,
           OUT_e_brkOn              := "I_MMI_SR".e_brk_on_fail,
           OUT_e_brkOff             := "I_MMI_SR".e_brk_off_fail,
           OUT_e_brkOnOff           := "I_MMI_SR".e_brk_onOff_fail,
           OUT_e_brkTrip            := "I_MMI_SR".e_brk_trip,
           OUT_e_synTime            := "I_MMI_SR".e_SynchrTime_Fail,
           OUT_e_StdbyStart         := "I_MMI_SR".e_StStart,
           OUT_e_ShoreActive        := "I_MMI_SR".e_GenBrk_ShoreConn,
           OUT_ind_ready            := "I_MMI_SR".a_GclseCriteria,
           OUT_ind_line1_stat       := "I_MMI_SR".a_GenSet_stat_ind,
           out_ind_line2_var        := "I_MMI_SR".a_GenSet_stat_var);
_007: NOP   0;
NETWORK
TITLE =Signal "command output 'tie breaker A close'"
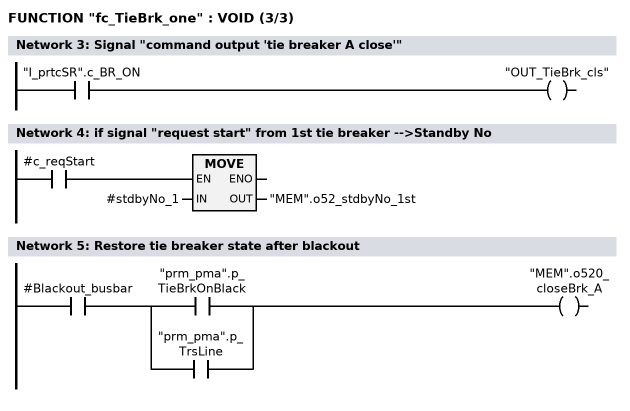
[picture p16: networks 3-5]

      U     "I_prtcSR".c_BR_ON;
      =     "OUT_TieBrk_cls";
NETWORK
TITLE =if signal "request start" from 1st tie breaker -->Standby No

      U     #c_reqStart;
      SPBNB _00b;
      L     #stdbyNo_1;
      T     "MEM".o52_stdbyNo_1st;
_00b: NOP   0;
NETWORK
TITLE =Restore tie breaker state after blackout

      U     #Blackout_busbar;
      U(    ;
      O     "prm_pma".p_TieBrkOnBlack;
      O     "prm_pma".p_TrsLine;
      )     ;
      =     "MEM".o520_closeBrk_A;
NETWORK
TITLE =Blocking tie breaker open if no diesel on busbar
//If this tie breaker the breaker between MSB and ESB in this case is this
//feature
//activated.
      L     #cfgBusbar;
      SLD   4;
      T     #total_CfgBusbar;

//Received commands from Gen 1 -13, EG, TieBrk 1-4, Shore1,2 (D38.2) <OR>
      CALL "fc_95_fdbHndl" (
           IN_off                   := B#16#8,
           IN_mask                  := B#16#FB,//bit0,1,3-7:AND ; bit2: OR
           IN_release               := #total_CfgBusbar,
           OUT_fdb                  := LB    12);//received MPI commands (byte 8)

      UN    #f_brk_clse_tb;
      U     "prm_pma".p_TrsLine;
      =     "MEM".o520_blockTBopn;
END_FUNCTION




